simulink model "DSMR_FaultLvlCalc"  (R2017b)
settings: Solver=FixedStepDiscrete  StartTime=0.0  StopTime=10.0  FixedStep=0.02  RelTol=1e-3  EnableMultiTasking=on
undefined symbols (not defined in the file): bin2dec, BMS_DSMR_FaultLvlCalc, Delay, Delay1, DFES_Cls_DFC_638LinCommErr_C, DFES_Cls_DFC_AcDischgFobd_C, DFES_Cls_DFC_AChgFobd_C, DFES_Cls_DFC_AChgHVOffTmt_C, DFES_Cls_DFC_AChgHVOnTmt_C, DFES_Cls_DFC_AChgingErr_C, DFES_Cls_DFC_AChgLckTmt_C, DFES_Cls_DFC_AChgPileRdyTmt_C, DFES_Cls_DFC_AChgRdyPndiTmt_C, DFES_Cls_DFC_AChgRdyTmt_C, DFES_Cls_DFC_AChgS2ClsdTmt_C, DFES_Cls_DFC_AChgUnlckTmt_C, DFES_Cls_DFC_AChrgCnntErr_C, DFES_Cls_DFC_AChrgCurrMish_C, DFES_Cls_DFC_AChrgPortOvrTemp_C, DFES_Cls_DFC_AChrgVoltMish_C, DFES_Cls_DFC_AFEAdcRelatedErr_C, DFES_Cls_DFC_AFECellTempUpdErr_C, DFES_Cls_DFC_AFECellVoltLineOpen_C, DFES_Cls_DFC_AFECellVoltUpdErr_C, DFES_Cls_DFC_AFEComLost_C, DFES_Cls_DFC_AFEDiagModeExitErr_C, DFES_Cls_DFC_AFEGpioLineOpen_C, DFES_Cls_DFC_AFEOtherErr_C, DFES_Cls_DFC_AFEResetFlt_C, DFES_Cls_DFC_AFESampleErr_C, DFES_Cls_DFC_AFESplyFlt_C, DFES_Cls_DFC_AFETempHighFlt_C, DFES_Cls_DFC_APlusChk_C, DFES_Cls_DFC_BalCirOpenFlt_C, DFES_Cls_DFC_BalCirShortFlt_C, DFES_Cls_DFC_BalStuckMax_C, DFES_Cls_DFC_BalStuckMin_C, DFES_Cls_DFC_BalTempHighFlt_C, DFES_Cls_DFC_BattCurrMismatchErr_C, DFES_Cls_DFC_BattHVMsgTmt_C, DFES_Cls_DFC_BattSohChk_C, DFES_Cls_DFC_BattTAlrmMax_C, DFES_Cls_DFC_BattTAlrmMin_C, DFES_Cls_DFC_BattTCnstMax_C, DFES_Cls_DFC_BattTempVldMax_C, DFES_Cls_DFC_BattTempVldMin_C, DFES_Cls_DFC_BattTFaultMax_C, DFES_Cls_DFC_BattTFaultMin_C, DFES_Cls_DFC_BattTGradtMax_C, DFES_Cls_DFC_BattTHopMax_C, DFES_Cls_DFC_BattTWarnMax_C, DFES_Cls_DFC_BattTWarnMin_C, DFES_Cls_DFC_BattUNpl_C, DFES_Cls_DFC_BattVoltHiMax_C, DFES_Cls_DFC_BattVoltLoMin_C, DFES_Cls_DFC_BattVoltRngErr_C, DFES_Cls_DFC_BattVoltVld_C, DFES_Cls_DFC_BMSSplyPwrAbnToCAB_C, DFES_Cls_DFC_BMSSplyPwrAbnToLem_C, DFES_Cls_DFC_BoardTempTmt_C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
libraries: simulink x535
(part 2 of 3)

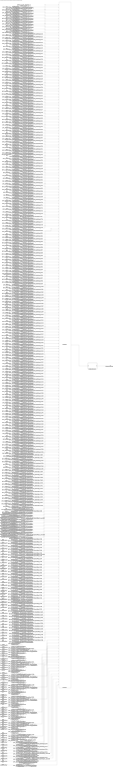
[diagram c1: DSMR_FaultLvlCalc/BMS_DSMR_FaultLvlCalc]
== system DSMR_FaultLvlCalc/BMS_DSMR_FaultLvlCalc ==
  DFC_CurrRngErr : Inport
  DFC_BattVoltRngErr : Inport  Port=2
  DFC_BattHVMsgTmt : Inport  Port=3
  DFC_BusHVMsgTmt : Inport  Port=4
  DFC_638LinCommErr : Inport  Port=5
  DFC_CellTempTmt : Inport  Port=6
  DFC_CellVoltTmt : Inport  Port=7
  DFC_InCanBusOff : Inport  Port=8
  DFC_VeCanBusOff : Inport  Port=9
  DFC_Msg2A3Tmt : Inport  Port=10
  DFC_RcMsg2A3Mis : Inport  Port=11
  DFC_ChkSumMsg2A3Err : Inport  Port=12
  DFC_RcMsg2A5Mis : Inport  Port=13
  DFC_RcMsg2A7Mis : Inport  Port=14
  DFC_CrashNpl : Inport  Port=15
  DFC_FuseNpl : Inport  Port=16
  DFC_Kl30cVoltLoErr : Inport  Port=17
  DFC_PosStuckMax : Inport  Port=18
  DFC_MPosStuckMin : Inport  Port=19
  DFC_MNegStuckMax : Inport  Port=20
  DFC_MNegStuckMin : Inport  Port=21
  DFC_PrStuckMin : Inport  Port=22
  DFC_DChrgPosStuckMax : Inport  Port=23
  DFC_DChrgPosStuckMin : Inport  Port=24
  DFC_DChrgNegStuckMax : Inport  Port=25
  DFC_DChrgNegStuckMin : Inport  Port=26
  DFC_HvPwrUpFail : Inport  Port=27
  DFC_DChrgPwrUpFail : Inport  Port=28
  DFC_BattTAlrmMax : Inport  Port=29
  DFC_BattTFaultMax : Inport  Port=30
  DFC_BattTAlrmMin : Inport  Port=31
  DFC_BattTFaultMin : Inport  Port=32
  DFC_BattTempVldMin : Inport  Port=33
  DFC_BattTCnstMax : Inport  Port=34
  DFC_BattTGradtMax : Inport  Port=35
  DFC_CellVoltAlrmMax : Inport  Port=36
  DFC_CellVoltFaultMax : Inport  Port=37
  DFC_CellVoltFusfMax : Inport  Port=38
  DFC_CellVoltAlrmMin : Inport  Port=39
  DFC_CellVoltFusfMin : Inport  Port=40
  DFC_CellVoltFaultMin : Inport  Port=41
  DFC_CellVoltVldMin : Inport  Port=42
  DFC_CellVoltNpl : Inport  Port=43
  DFC_Msg2E6Tmt : Inport  Port=44
  DFC_RcMsg2E6Mis : Inport  Port=45
  DFC_ChkSumMsg2E6Err : Inport  Port=46
  DFC_RcMsg2E1Mis : Inport  Port=47
  DFC_ChkSumMsg2E1Err : Inport  Port=48
  DFC_DcCanBusOff : Inport  Port=49
  DFC_DChrgTCnntMax : Inport  Port=50
  DFC_ChrgOCNpl : Inport  Port=51
  DFC_DisChOCNpl : Inport  Port=52
  DFC_BattVoltHiMax : Inport  Port=53
  DFC_BattVoltLoMin : Inport  Port=54
  DFC_ThmRnwy : Inport  Port=55
  DFC_AChrgPortOvrTemp : Inport  Port=56
  DFC_CurrOffsPlaus : Inport  Port=57
  DFC_CurrStukPlaus : Inport  Port=58
  DFC_CurrChrgPlaus : Inport  Port=59
  DFC_BattUNpl : Inport  Port=60
  DFC_BattVoltVld : Inport  Port=61
  DFC_PackUNpl : Inport  Port=62
  DFC_PackVoltVld : Inport  Port=63
  DFC_DChrgUNpl : Inport  Port=64
  DFC_DChrgVoltVld : Inport  Port=65
  DFC_BoardTempTmt : Inport  Port=66
  DFC_HvilMax : Inport  Port=67
  DFC_HvilMin : Inport  Port=68
  DFC_HvilSig : Inport  Port=69
  DFC_ChkSumMsg050Err : Inport  Port=70
  DFC_RcMsg050Mis : Inport  Port=71
  DFC_CrashHwNpl : Inport  Port=72
  DFC_IsoChkLv1 : Inport  Port=73
  DFC_IsoChkLv2 : Inport  Port=74
  DFC_InsResValdFault : Inport  Port=75
  DFC_Kl30OutRngErr : Inport  Port=76
  DFC_Kl30VoltLoErr : Inport  Port=77
  DFC_Kl30VoltHiErr : Inport  Port=78
  DFC_EepReadErr : Inport  Port=79
  DFC_BalStuckMax : Inport  Port=80
  DFC_BalStuckMin : Inport  Port=81
  DFC_CSCPwrSpyHiErr : Inport  Port=82
  DFC_CSCPwrSpyLoErr : Inport  Port=83
  DFC_CmcBordOTMax : Inport  Port=84
  DFC_BattTWarnMax : Inport  Port=85
  DFC_BattTWarnMin : Inport  Port=86
  DFC_BattTempVldMax : Inport  Port=87
  DFC_BattTHopMax : Inport  Port=88
  DFC_CellVoltRngHiErr : Inport  Port=89
  DFC_CellVoltRngLoErr : Inport  Port=90
  DFC_CellVoltWarnMax : Inport  Port=91
  DFC_CellVoltWarnMin : Inport  Port=92
  DFC_CellVoltVldMax : Inport  Port=93
  DFC_AChrgCurrMish : Inport  Port=94
  DFC_DChrgCurrMish : Inport  Port=95
  DFC_DChrgLowTempCurrMish : Inport  Port=96
  DFC_AChrgVoltMish : Inport  Port=97
  DFC_DChrgVoltMish : Inport  Port=98
  DFC_DChrgBattTMin : Inport  Port=99
  DFC_CC2Chk : Inport  Port=100
  DFC_APlusChk : Inport  Port=101
  DFC_DChrgMsgTmt : Inport  Port=102
  DFC_DChrgTNegElecMax : Inport  Port=103
  DFC_DChrgTNegElecMin : Inport  Port=104
  DFC_DChrgTNegElecSig : Inport  Port=105
  DFC_DChrgTPosElecMax : Inport  Port=106
  DFC_DChrgTPosElecMin : Inport  Port=107
  DFC_DChrgTPosElecSig : Inport  Port=108
  DFC_CcuSelfChkErr : Inport  Port=109
  DFC_ChrgOCMin : Inport  Port=110
  DFC_ChrgOCMax : Inport  Port=111
  DFC_DisChOCMin : Inport  Port=112
  DFC_DisChOCMax : Inport  Port=113
  DFC_SocRngLoMax : Inport  Port=114
  DFC_SocRngLoMin : Inport  Port=115
  DFC_SocRngHiMax : Inport  Port=116
  DFC_SocRngHiMin : Inport  Port=117
  DFC_InClntOverTmp : Inport  Port=118
  DFC_OutClntOverTmp : Inport  Port=119
  DFC_ClntDsTElecMax : Inport  Port=120
  DFC_ClntDsTElecMin : Inport  Port=121
  DFC_ClntDsTElecSig : Inport  Port=122
  DFC_ClntUsTElecMax : Inport  Port=123
  DFC_ClntUsTElecMin : Inport  Port=124
  DFC_ClntUsTElecSig : Inport  Port=125
  DFC_CoolPerfPlaus : Inport  Port=126
  DFC_HtgPerfPlaus : Inport  Port=127
  DFC_DChrgFobd : Inport  Port=128
  DFC_DChrgHvOnFail : Inport  Port=129
  DFC_AChgHVOnTmt : Inport  Port=130
  DFC_AChgHVOffTmt : Inport  Port=131
  DFC_AChgS2ClsdTmt : Inport  Port=132
  DFC_DChrgStakeErr : Inport  Port=133
  DFC_DChrgStkVoltErr : Inport  Port=134
  DFC_DChrgStkCurrErr : Inport  Port=135
  DFC_AChgPileRdyTmt : Inport  Port=136
  DFC_DChrgCHMTmt : Inport  Port=137
  DFC_DChrgCRMTmt : Inport  Port=138
  DFC_DChrgCMLTmt : Inport  Port=139
  DFC_DChrgCROTmt : Inport  Port=140
  DFC_DChrgCCSTmt : Inport  Port=141
  DFC_DChrgCSTTmt : Inport  Port=142
  DFC_DChrgCSDTmt : Inport  Port=143
  DFC_DChrgParaChk : Inport  Port=144
  DFC_DChrgCableChk : Inport  Port=145
  DFC_DChrgSLACTOut : Inport  Port=146
  DFC_DChrgCnntErr : Inport  Port=147
  DFC_DChrgLckErr : Inport  Port=148
  DFC_AChrgCnntErr : Inport  Port=149
  DFC_AChgLckTmt : Inport  Port=150
  DFC_AChgRdyPndiTmt : Inport  Port=151
  DFC_AChgRdyTmt : Inport  Port=152
  DFC_AChgingErr : Inport  Port=153
  DFC_AChgUnlckTmt : Inport  Port=154
  DFC_AChgFobd : Inport  Port=155
  DFC_SocValJmp : Inport  Port=156
  DFC_ChrgCmuLost : Inport  Port=157
  DFC_DisChrgCmuLost : Inport  Port=158
  DFC_Msg130Tmt : Inport  Port=159
  DFC_Msg2E1Tmt : Inport  Port=160
  DFC_Msg2EBTmt : Inport  Port=161
  DFC_MsgCABTmt : Inport  Port=162
  DFC_Msg0B5Tmt : Inport  Port=163
  DFC_ObcTmt : Inport  Port=164
  DFC_VcuTmt : Inport  Port=165
  DFC_Msg2A7Tmt : Inport  Port=166
  DFC_Msg2A5Tmt : Inport  Port=167
  DFC_Msg2ADTmt : Inport  Port=168
  DFC_Msg2BBTmt : Inport  Port=169
  DFC_Msg2DFTmt : Inport  Port=170
  DFC_Msg3AATmt : Inport  Port=171
  DFC_Msg050Tmt : Inport  Port=172
  DFC_Msg2F1Tmt : Inport  Port=173
  DFC_Msg195Tmt : Inport  Port=174
  DFC_Msg37FTmt : Inport  Port=175
  DFC_Msg28CTmt : Inport  Port=176
  DFC_Msg17DTmt : Inport  Port=177
  DFC_HwCurrElecSCG : Inport  Port=178
  DFC_HwCurrElecSCP : Inport  Port=179
  DFC_CABErr : Inport  Port=180
  DFC_BattCurrMismatchErr : Inport  Port=181
  GaCFM_AFEComLost_flg : Inport  Port=182
  GaCFM_AFECellVoltUpdErr_flg : Inport  Port=183
  GaCFM_AFECellTempUpdErr_flg : Inport  Port=184
  GaCFM_AFESampleErr_flg : Inport  Port=185
  GaCFM_AFECellVoltLineOpen_flg : Inport  Port=186
  GaCFM_AFEGpioLineOpen_flg : Inport  Port=187
  GaCFM_AFEAdcRelatedErr_flg : Inport  Port=188
  GaCFM_AFEDiagModeExitErr_flg : Inport  Port=189
  GaCFM_AFEOtherErr_flg : Inport  Port=190
  DFC_AcDischgFobd : Inport  Port=191
  DFC_BalCirOpenFlt : Inport  Port=192
  DFC_BalCirShortFlt : Inport  Port=193
  DFC_BalTempHighFlt : Inport  Port=194
  DFC_HVSmplComFlt : Inport  Port=195
  DFC_HVSmplSigErr : Inport  Port=196
  DFC_HVSmplSplyFlt : Inport  Port=197
  DFC_CABVoltOutOfRng : Inport  Port=198
  DFC_CABDevFlt : Inport  Port=199
  DFC_BMSSplyPwrAbnToLem : Inport  Port=200
  DFC_BMSSplyPwrAbnToCAB : Inport  Port=201
  DFC_NVMReadError : Inport  Port=202
  DFC_KL30Shutdown : Inport  Port=203
  DFC_MCUResetFlt : Inport  Port=204
  DFC_BattSohChk : Inport  Port=205
  DFC_CalCANBusOff : Inport  Port=206
  DFC_ThmRnwyWarn : Inport  Port=207
  DFC_PchgOvrCurrFlt : Inport  Port=208
  DFC_SBCSplyPwrOvrVolt : Inport  Port=209
  DFC_SBCSplyPwrUnderVolt : Inport  Port=210
  DFC_SBCSplyPwrOvrCurr : Inport  Port=211
  DFC_CrashChkHwFrqAbnorm : Inport  Port=212
  DFC_CrashChkHwDutyAbnorm : Inport  Port=213
  DFC_AFETempHighFlt : Inport  Port=214
  DFC_EVCCDevFlt : Inport  Port=215
  DFC_EVCCSplyPwrFlt : Inport  Port=216
  DFC_EVCCVehComFlt : Inport  Port=217
  DFC_EVCCPileComFlt : Inport  Port=218
  DFC_EVCCVehHwFlt : Inport  Port=219
  DFC_EVCCPileHwFlt : Inport  Port=220
  DFC_IsoS1SwStuckOpen : Inport  Port=221
  DFC_IsoS1SwStuckClsd : Inport  Port=222
  DFC_IsoS2SwStuckOpen : Inport  Port=223
  DFC_IsoS2SwStuckClsd : Inport  Port=224
  DFC_IsoS3SwStuckOpen : Inport  Port=225
  DFC_IsoS3SwStuckClsd : Inport  Port=226
  DFC_AFEResetFlt : Inport  Port=227
  DFC_AFESplyFlt : Inport  Port=228
  DFC_PreHeatErr : Inport  Port=229
  DFC_PreHeatVcuReqTmt : Inport  Port=230
  DFC_PreHeatObcStatusErr : Inport  Port=231
  DFC_PreHeatPtcErr : Inport  Port=232
  DFC_MPosRlyDrvScb : Inport  Port=233
  DFC_MPosRlyDrvScg : Inport  Port=234
  DFC_MPosRlyDrvOL : Inport  Port=235
  DFC_MposRlyDrvOvrCurr : Inport  Port=236
  DFC_MPosRlyDrvFault : Inport  Port=237
  DFC_MNegRlyDrvScb : Inport  Port=238
  DFC_MNegRlyDrvScg : Inport  Port=239
  DFC_MNegRlyDrvOL : Inport  Port=240
  DFC_MNegRlyDrvOvrCurr : Inport  Port=241
  DFC_MNegRlyDrvFault : Inport  Port=242
  DFC_DcPosRlyDrvScb : Inport  Port=243
  DFC_DcPosRlyDrvScg : Inport  Port=244
  DFC_DcPosRlyDrvOL : Inport  Port=245
  DFC_DChrgPosRlyDrvOvrCurr : Inport  Port=246
  DFC_DcPosRlyDrvFault : Inport  Port=247
  DFC_DcNegRlyDrvScb : Inport  Port=248
  DFC_DcNegRlyDrvScg : Inport  Port=249
  DFC_DcNegRlyDrvOL : Inport  Port=250
  DFC_DChrgNegRlyDrvOvrCurr : Inport  Port=251
  DFC_DcNegRlyDrvFault : Inport  Port=252
  DFC_PreRlyDrvScb : Inport  Port=253
  DFC_PreRlyDrvScg : Inport  Port=254
  DFC_PreRlyDrvOL : Inport  Port=255
  DFC_PrRlyDrvOvrCurr : Inport  Port=256
  DFC_CellTAlrmMax : Inport  Port=257
  DFC_CellTFaultMax : Inport  Port=258
  DFC_CellTAlrmMin : Inport  Port=259
  DFC_CellTFaultMin : Inport  Port=260
  DFC_CellTempVldMin : Inport  Port=261
  DFC_CellTCnstMax : Inport  Port=262
  DFC_CellTGradtMax : Inport  Port=263
  DFC_CellTWarnMax : Inport  Port=264
  DFC_CellTWarnMin : Inport  Port=265
  DFC_CellTempVldMax : Inport  Port=266
  DFC_CellTHopMax : Inport  Port=267
  DFC_TwoCurrSnsrFlt : Inport  Port=268
  DFC_ThmRnwyAlarm : Inport  Port=269
  DFC_ChkSumMsg2A5Err : Inport  Port=270
  DFC_ChkSumMsg2A7Err : Inport  Port=271
  DFC_DchrgIsoChkLv1 : Inport  Port=272
  DFC_DchrgIsoChkLv2 : Inport  Port=273
  DFC_HVOffIsoChkLv1 : Inport  Port=274
  DFC_HVOffIsoChkLv2 : Inport  Port=275
  DFC_PackCrntSaf : Inport  Port=276
  DFC_BattUNpl_{1..267} (267 alike) : simulink/Logic and Bit Operations/Bitwise Operator  logicop=AND  UseBitMask=on  BitMask=bin2dec('00011000')  BitMaskRealWorld=Stored Integer
  DFC_BattUNpl_1_compare{,1..266} (267 alike) : simulink/Logic and Bit Operations/Compare To Constant  relop===  const=24  OutDataTypeStr=boolean
  DFC_BattUNpl_applied{,1..243} (244 alike) : Switch  Criteria=u2 > Threshold
  DFES_Cls_DFC_BattUNpl_C : Constant  Value=DFES_Cls_DFC_CurrRngErr_C
  DFES_Cls_DFC_BattUNpl_C1 : Constant  Value=DFES_Cls_DFC_BattVoltRngErr_C
  DFES_Cls_DFC_BattUNpl_C10 : Constant  Value=DFES_Cls_DFC_RcMsg2A3Mis_C
  DFES_Cls_DFC_BattUNpl_C100 : Constant  Value=DFES_Cls_DFC_APlusChk_C
  DFES_Cls_DFC_BattUNpl_C101 : Constant  Value=DFES_Cls_DFC_DChrgMsgTmt_C
  DFES_Cls_DFC_BattUNpl_C102 : Constant  Value=DFES_Cls_DFC_DChrgTNegElecMax_C
  DFES_Cls_DFC_BattUNpl_C103 : Constant  Value=DFES_Cls_DFC_DChrgTNegElecMin_C
  DFES_Cls_DFC_BattUNpl_C104 : Constant  Value=DFES_Cls_DFC_DChrgTNegElecSig_C
  DFES_Cls_DFC_BattUNpl_C105 : Constant  Value=DFES_Cls_DFC_DChrgTPosElecMax_C
  DFES_Cls_DFC_BattUNpl_C106 : Constant  Value=DFES_Cls_DFC_DChrgTPosElecMin_C
  DFES_Cls_DFC_BattUNpl_C107 : Constant  Value=DFES_Cls_DFC_DChrgTPosElecSig_C
  DFES_Cls_DFC_BattUNpl_C108 : Constant  Value=DFES_Cls_DFC_CcuSelfChkErr_C
  DFES_Cls_DFC_BattUNpl_C109 : Constant  Value=DFES_Cls_DFC_ChrgOCMin_C
  DFES_Cls_DFC_BattUNpl_C11 : Constant  Value=DFES_Cls_DFC_ChkSumMsg2A3Err_C
  DFES_Cls_DFC_BattUNpl_C110 : Constant  Value=DFES_Cls_DFC_ChrgOCMax_C
  DFES_Cls_DFC_BattUNpl_C111 : Constant  Value=DFES_Cls_DFC_DisChOCMin_C
  DFES_Cls_DFC_BattUNpl_C112 : Constant  Value=DFES_Cls_DFC_DisChOCMax_C
  DFES_Cls_DFC_BattUNpl_C113 : Constant  Value=DFES_Cls_DFC_SocRngLoMax_C
  DFES_Cls_DFC_BattUNpl_C114 : Constant  Value=DFES_Cls_DFC_SocRngLoMin_C
  DFES_Cls_DFC_BattUNpl_C115 : Constant  Value=DFES_Cls_DFC_SocRngHiMax_C
  DFES_Cls_DFC_BattUNpl_C116 : Constant  Value=DFES_Cls_DFC_SocRngHiMin_C
  DFES_Cls_DFC_BattUNpl_C117 : Constant  Value=DFES_Cls_DFC_InClntOverTmp_C
  DFES_Cls_DFC_BattUNpl_C118 : Constant  Value=DFES_Cls_DFC_OutClntOverTmp_C
  DFES_Cls_DFC_BattUNpl_C119 : Constant  Value=DFES_Cls_DFC_ClntDsTElecMax_C
  DFES_Cls_DFC_BattUNpl_C12 : Constant  Value=DFES_Cls_DFC_RcMsg2A5Mis_C
  DFES_Cls_DFC_BattUNpl_C120 : Constant  Value=DFES_Cls_DFC_ClntDsTElecMin_C
  DFES_Cls_DFC_BattUNpl_C121 : Constant  Value=DFES_Cls_DFC_ClntDsTElecSig_C
  DFES_Cls_DFC_BattUNpl_C122 : Constant  Value=DFES_Cls_DFC_ClntUsTElecMax_C
  DFES_Cls_DFC_BattUNpl_C123 : Constant  Value=DFES_Cls_DFC_ClntUsTElecMin_C
  DFES_Cls_DFC_BattUNpl_C124 : Constant  Value=DFES_Cls_DFC_ClntUsTElecSig_C
  DFES_Cls_DFC_BattUNpl_C125 : Constant  Value=DFES_Cls_DFC_CoolPerfPlaus_C
  DFES_Cls_DFC_BattUNpl_C126 : Constant  Value=DFES_Cls_DFC_HtgPerfPlaus_C
  DFES_Cls_DFC_BattUNpl_C127 : Constant  Value=DFES_Cls_DFC_DChrgFobd_C
  DFES_Cls_DFC_BattUNpl_C128 : Constant  Value=DFES_Cls_DFC_DChrgHvOnFail_C
  DFES_Cls_DFC_BattUNpl_C129 : Constant  Value=DFES_Cls_DFC_AChgHVOnTmt_C
  DFES_Cls_DFC_BattUNpl_C13 : Constant  Value=DFES_Cls_DFC_RcMsg2A7Mis_C
  DFES_Cls_DFC_BattUNpl_C130 : Constant  Value=DFES_Cls_DFC_AChgHVOffTmt_C
  DFES_Cls_DFC_BattUNpl_C131 : Constant  Value=DFES_Cls_DFC_AChgS2ClsdTmt_C
  DFES_Cls_DFC_BattUNpl_C132 : Constant  Value=DFES_Cls_DFC_DChrgStakeErr_C
  DFES_Cls_DFC_BattUNpl_C133 : Constant  Value=DFES_Cls_DFC_DChrgStkVoltErr_C
  DFES_Cls_DFC_BattUNpl_C134 : Constant  Value=DFES_Cls_DFC_DChrgStkCurrErr_C
  DFES_Cls_DFC_BattUNpl_C135 : Constant  Value=DFES_Cls_DFC_AChgPileRdyTmt_C
  DFES_Cls_DFC_BattUNpl_C136 : Constant  Value=DFES_Cls_DFC_DChrgCHMTmt_C
  DFES_Cls_DFC_BattUNpl_C137 : Constant  Value=DFES_Cls_DFC_DChrgCRMTmt_C
  DFES_Cls_DFC_BattUNpl_C138 : Constant  Value=DFES_Cls_DFC_DChrgCMLTmt_C
  DFES_Cls_DFC_BattUNpl_C139 : Constant  Value=DFES_Cls_DFC_DChrgCROTmt_C
  DFES_Cls_DFC_BattUNpl_C14 : Constant  Value=DFES_Cls_DFC_CrashNpl_C
  DFES_Cls_DFC_BattUNpl_C140 : Constant  Value=DFES_Cls_DFC_DChrgCCSTmt_C
  DFES_Cls_DFC_BattUNpl_C141 : Constant  Value=DFES_Cls_DFC_DChrgCSTTmt_C
  DFES_Cls_DFC_BattUNpl_C142 : Constant  Value=DFES_Cls_DFC_DChrgCSDTmt_C
  DFES_Cls_DFC_BattUNpl_C143 : Constant  Value=DFES_Cls_DFC_DChrgParaChk_C
  DFES_Cls_DFC_BattUNpl_C144 : Constant  Value=DFES_Cls_DFC_DChrgCableChk_C
  DFES_Cls_DFC_BattUNpl_C145 : Constant  Value=DFES_Cls_DFC_DChrgSLACTOut_C
  DFES_Cls_DFC_BattUNpl_C146 : Constant  Value=DFES_Cls_DFC_DChrgCnntErr_C
  DFES_Cls_DFC_BattUNpl_C147 : Constant  Value=DFES_Cls_DFC_DChrgLckErr_C
  DFES_Cls_DFC_BattUNpl_C148 : Constant  Value=DFES_Cls_DFC_AChrgCnntErr_C
  DFES_Cls_DFC_BattUNpl_C149 : Constant  Value=DFES_Cls_DFC_AChgLckTmt_C
  DFES_Cls_DFC_BattUNpl_C15 : Constant  Value=DFES_Cls_DFC_FuseNpl_C
  DFES_Cls_DFC_BattUNpl_C150 : Constant  Value=DFES_Cls_DFC_AChgRdyPndiTmt_C
  DFES_Cls_DFC_BattUNpl_C151 : Constant  Value=DFES_Cls_DFC_AChgRdyTmt_C
  DFES_Cls_DFC_BattUNpl_C152 : Constant  Value=DFES_Cls_DFC_AChgingErr_C
  DFES_Cls_DFC_BattUNpl_C153 : Constant  Value=DFES_Cls_DFC_AChgUnlckTmt_C
  DFES_Cls_DFC_BattUNpl_C154 : Constant  Value=DFES_Cls_DFC_AChgFobd_C
  DFES_Cls_DFC_BattUNpl_C155 : Constant  Value=DFES_Cls_DFC_SocValJmp_C
  DFES_Cls_DFC_BattUNpl_C156 : Constant  Value=DFES_Cls_DFC_ChrgCmuLost_C
  DFES_Cls_DFC_BattUNpl_C157 : Constant  Value=DFES_Cls_DFC_DisChrgCmuLost_C
  DFES_Cls_DFC_BattUNpl_C158 : Constant  Value=DFES_Cls_DFC_Msg130Tmt_C
  DFES_Cls_DFC_BattUNpl_C159 : Constant  Value=DFES_Cls_DFC_Msg2E1Tmt_C
  DFES_Cls_DFC_BattUNpl_C16 : Constant  Value=DFES_Cls_DFC_Kl30cVoltLoErr_C
  DFES_Cls_DFC_BattUNpl_C160 : Constant  Value=DFES_Cls_DFC_Msg2EBTmt_C
  DFES_Cls_DFC_BattUNpl_C161 : Constant  Value=DFES_Cls_DFC_MsgCABTmt_C
  DFES_Cls_DFC_BattUNpl_C162 : Constant  Value=DFES_Cls_DFC_Msg0B5Tmt_C
  DFES_Cls_DFC_BattUNpl_C163 : Constant  Value=DFES_Cls_DFC_ObcTmt_C
  DFES_Cls_DFC_BattUNpl_C164 : Constant  Value=DFES_Cls_DFC_VcuTmt_C
  DFES_Cls_DFC_BattUNpl_C165 : Constant  Value=DFES_Cls_DFC_Msg2A7Tmt_C
  DFES_Cls_DFC_BattUNpl_C166 : Constant  Value=DFES_Cls_DFC_Msg2A5Tmt_C
  DFES_Cls_DFC_BattUNpl_C167 : Constant  Value=DFES_Cls_DFC_Msg2ADTmt_C
  DFES_Cls_DFC_BattUNpl_C168 : Constant  Value=DFES_Cls_DFC_Msg2BBTmt_C
  DFES_Cls_DFC_BattUNpl_C169 : Constant  Value=DFES_Cls_DFC_Msg2DFTmt_C
  DFES_Cls_DFC_BattUNpl_C17 : Constant  Value=DFES_Cls_DFC_PosStuckMax_C
  DFES_Cls_DFC_BattUNpl_C170 : Constant  Value=DFES_Cls_DFC_Msg3AATmt_C
  DFES_Cls_DFC_BattUNpl_C171 : Constant  Value=DFES_Cls_DFC_Msg050Tmt_C
  DFES_Cls_DFC_BattUNpl_C172 : Constant  Value=DFES_Cls_DFC_Msg2F1Tmt_C
  DFES_Cls_DFC_BattUNpl_C173 : Constant  Value=DFES_Cls_DFC_Msg37FTmt_C
  DFES_Cls_DFC_BattUNpl_C174 : Constant  Value=DFES_Cls_DFC_Msg28CTmt_C
  DFES_Cls_DFC_BattUNpl_C175 : Constant  Value=DFES_Cls_DFC_Msg17DTmt_C
  DFES_Cls_DFC_BattUNpl_C176 : Constant  Value=DFES_Cls_DFC_HwCurrElecSCG_C
  DFES_Cls_DFC_BattUNpl_C177 : Constant  Value=DFES_Cls_DFC_HwCurrElecSCP_C
  DFES_Cls_DFC_BattUNpl_C178 : Constant  Value=DFES_Cls_DFC_CABErr_C
  DFES_Cls_DFC_BattUNpl_C179 : Constant  Value=DFES_Cls_DFC_BattCurrMismatchErr_C
  DFES_Cls_DFC_BattUNpl_C18 : Constant  Value=DFES_Cls_DFC_MPosStuckMin_C
  DFES_Cls_DFC_BattUNpl_C180 : Constant  Value=DFES_Cls_DFC_Msg195Tmt_C
  DFES_Cls_DFC_BattUNpl_C181 : Constant  Value=DFES_Cls_DFC_AFEComLost_C
  DFES_Cls_DFC_BattUNpl_C182 : Constant  Value=DFES_Cls_DFC_AFECellVoltUpdErr_C
  DFES_Cls_DFC_BattUNpl_C183 : Constant  Value=DFES_Cls_DFC_AFECellTempUpdErr_C
  DFES_Cls_DFC_BattUNpl_C184 : Constant  Value=DFES_Cls_DFC_AFESampleErr_C
  DFES_Cls_DFC_BattUNpl_C185 : Constant  Value=DFES_Cls_DFC_AFECellVoltLineOpen_C
  DFES_Cls_DFC_BattUNpl_C186 : Constant  Value=DFES_Cls_DFC_AFEGpioLineOpen_C
  DFES_Cls_DFC_BattUNpl_C187 : Constant  Value=DFES_Cls_DFC_AFEAdcRelatedErr_C
  DFES_Cls_DFC_BattUNpl_C188 : Constant  Value=DFES_Cls_DFC_AFEDiagModeExitErr_C
  DFES_Cls_DFC_BattUNpl_C189 : Constant  Value=DFES_Cls_DFC_AFEOtherErr_C
  DFES_Cls_DFC_BattUNpl_C19 : Constant  Value=DFES_Cls_DFC_MNegStuckMax_C
  DFES_Cls_DFC_BattUNpl_C190 : Constant  Value=DFES_Cls_DFC_AcDischgFobd_C
  DFES_Cls_DFC_BattUNpl_C191 : Constant  Value=DFES_Cls_DFC_BalCirOpenFlt_C
  DFES_Cls_DFC_BattUNpl_C192 : Constant  Value=DFES_Cls_DFC_BalCirShortFlt_C
  DFES_Cls_DFC_BattUNpl_C193 : Constant  Value=DFES_Cls_DFC_BalTempHighFlt_C
  DFES_Cls_DFC_BattUNpl_C194 : Constant  Value=DFES_Cls_DFC_HVSmplComFlt_C
  DFES_Cls_DFC_BattUNpl_C195 : Constant  Value=DFES_Cls_DFC_HVSmplSigErr_C
  DFES_Cls_DFC_BattUNpl_C196 : Constant  Value=DFES_Cls_DFC_HVSmplSplyFlt_C
  DFES_Cls_DFC_BattUNpl_C197 : Constant  Value=DFES_Cls_DFC_CABVoltOutOfRng_C
  DFES_Cls_DFC_BattUNpl_C198 : Constant  Value=DFES_Cls_DFC_CABDevFlt_C
  DFES_Cls_DFC_BattUNpl_C199 : Constant  Value=DFES_Cls_DFC_BMSSplyPwrAbnToLem_C
  DFES_Cls_DFC_BattUNpl_C2 : Constant  Value=DFES_Cls_DFC_BattHVMsgTmt_C
  DFES_Cls_DFC_BattUNpl_C20 : Constant  Value=DFES_Cls_DFC_MNegStuckMin_C
  DFES_Cls_DFC_BattUNpl_C200 : Constant  Value=DFES_Cls_DFC_BMSSplyPwrAbnToCAB_C
  DFES_Cls_DFC_BattUNpl_C201 : Constant  Value=DFES_Cls_DFC_NVMReadError_C
  DFES_Cls_DFC_BattUNpl_C202 : Constant  Value=DFES_Cls_DFC_KL30Shutdown_C
  DFES_Cls_DFC_BattUNpl_C203 : Constant  Value=DFES_Cls_DFC_MCUResetFlt_C
  DFES_Cls_DFC_BattUNpl_C204 : Constant  Value=DFES_Cls_DFC_BattSohChk_C
  DFES_Cls_DFC_BattUNpl_C205 : Constant  Value=DFES_Cls_DFC_CalCANBusOff_C
  DFES_Cls_DFC_BattUNpl_C206 : Constant  Value=DFES_Cls_DFC_ThmRnwyWarn_C
  DFES_Cls_DFC_BattUNpl_C207 : Constant  Value=DFES_Cls_DFC_PchgOvrCurrFlt_C
  DFES_Cls_DFC_BattUNpl_C208 : Constant  Value=DFES_Cls_DFC_SBCSplyPwrOvrVolt_C
  DFES_Cls_DFC_BattUNpl_C209 : Constant  Value=DFES_Cls_DFC_SBCSplyPwrUnderVolt_C
  DFES_Cls_DFC_BattUNpl_C21 : Constant  Value=DFES_Cls_DFC_PrStuckMin_C
  DFES_Cls_DFC_BattUNpl_C210 : Constant  Value=DFES_Cls_DFC_SBCSplyPwrOvrCurr_C
  DFES_Cls_DFC_BattUNpl_C211 : Constant  Value=DFES_Cls_DFC_CrashChkHwFrqAbnorm_C
  DFES_Cls_DFC_BattUNpl_C212 : Constant  Value=DFES_Cls_DFC_AFETempHighFlt_C
  DFES_Cls_DFC_BattUNpl_C213 : Constant  Value=DFES_Cls_DFC_CrashChkHwDutyAbnorm_C
  DFES_Cls_DFC_BattUNpl_C214 : Constant  Value=DFES_Cls_DFC_EVCCFlt_C
  DFES_Cls_DFC_BattUNpl_C215 : Constant  Value=DFES_Cls_DFC_IsoSwFlt_C
  DFES_Cls_DFC_BattUNpl_C216 : Constant  Value=DFES_Cls_DFC_AFEResetFlt_C
  DFES_Cls_DFC_BattUNpl_C217 : Constant  Value=DFES_Cls_DFC_AFESplyFlt_C
  DFES_Cls_DFC_BattUNpl_C218 : Constant  Value=DFES_Cls_DFC_PreHeatFlt_C
  DFES_Cls_DFC_BattUNpl_C219 : Constant  Value=DFES_Cls_DFC_MPosRlyDrv_C
  DFES_Cls_DFC_BattUNpl_C22 : Constant  Value=DFES_Cls_DFC_DChrgPosStuckMax_C
  DFES_Cls_DFC_BattUNpl_C220 : Constant  Value=DFES_Cls_DFC_MNegRlyDrv_C
  DFES_Cls_DFC_BattUNpl_C221 : Constant  Value=DFES_Cls_DFC_DCPosRlyDrv_C
  DFES_Cls_DFC_BattUNpl_C222 : Constant  Value=DFES_Cls_DFC_DCNegRlyDrv_C
  DFES_Cls_DFC_BattUNpl_C223 : Constant  Value=DFES_Cls_DFC_PrRlyDrv_C
  DFES_Cls_DFC_BattUNpl_C224 : Constant  Value=DFES_Cls_DFC_CellTAlrmMax_C
  DFES_Cls_DFC_BattUNpl_C225 : Constant  Value=DFES_Cls_DFC_CellTFaultMax_C
  DFES_Cls_DFC_BattUNpl_C226 : Constant  Value=DFES_Cls_DFC_CellTAlrmMin_C
  DFES_Cls_DFC_BattUNpl_C227 : Constant  Value=DFES_Cls_DFC_CellTFaultMin_C
  DFES_Cls_DFC_BattUNpl_C228 : Constant  Value=DFES_Cls_DFC_CellTempVldMin_C
  DFES_Cls_DFC_BattUNpl_C229 : Constant  Value=DFES_Cls_DFC_CellTCnstMax_C
  DFES_Cls_DFC_BattUNpl_C23 : Constant  Value=DFES_Cls_DFC_DChrgPosStuckMin_C
  DFES_Cls_DFC_BattUNpl_C230 : Constant  Value=DFES_Cls_DFC_CellTGradtMax_C
  DFES_Cls_DFC_BattUNpl_C231 : Constant  Value=DFES_Cls_DFC_CellTWarnMax_C
  DFES_Cls_DFC_BattUNpl_C232 : Constant  Value=DFES_Cls_DFC_CellTWarnMin_C
  DFES_Cls_DFC_BattUNpl_C233 : Constant  Value=DFES_Cls_DFC_CellTempVldMax_C
  DFES_Cls_DFC_BattUNpl_C234 : Constant  Value=DFES_Cls_DFC_CellTHopMax_C
  DFES_Cls_DFC_BattUNpl_C235 : Constant  Value=DFES_Cls_DFC_TwoCurrSnsrFlt_C
  DFES_Cls_DFC_BattUNpl_C236 : Constant  Value=DFES_Cls_DFC_ThmRnwyAlarm_C
  DFES_Cls_DFC_BattUNpl_C237 : Constant  Value=DFES_Cls_DFC_ChkSumMsg2A5Err_C
  DFES_Cls_DFC_BattUNpl_C238 : Constant  Value=DFES_Cls_DFC_ChkSumMsg2A7Err_C
  DFES_Cls_DFC_BattUNpl_C239 : Constant  Value=DFES_Cls_DFC_DchrgIsoChkLv1_C
  DFES_Cls_DFC_BattUNpl_C24 : Constant  Value=DFES_Cls_DFC_DChrgNegStuckMax_C
  DFES_Cls_DFC_BattUNpl_C240 : Constant  Value=DFES_Cls_DFC_DchrgIsoChkLv2_C
  DFES_Cls_DFC_BattUNpl_C241 : Constant  Value=DFES_Cls_DFC_HVOffIsoChkLv1_C
  DFES_Cls_DFC_BattUNpl_C242 : Constant  Value=DFES_Cls_DFC_HVOffIsoChkLv2_C
  DFES_Cls_DFC_BattUNpl_C243 : Constant  Value=DFES_Cls_DFC_PackCrntSaf_C
  DFES_Cls_DFC_BattUNpl_C25 : Constant  Value=DFES_Cls_DFC_DChrgNegStuckMin_C
  DFES_Cls_DFC_BattUNpl_C26 : Constant  Value=DFES_Cls_DFC_HvPwrUpFail_C
  DFES_Cls_DFC_BattUNpl_C27 : Constant  Value=DFES_Cls_DFC_DChrgPwrUpFail_C
  DFES_Cls_DFC_BattUNpl_C28 : Constant  Value=DFES_Cls_DFC_BattTAlrmMax_C
  DFES_Cls_DFC_BattUNpl_C29 : Constant  Value=DFES_Cls_DFC_BattTFaultMax_C
  DFES_Cls_DFC_BattUNpl_C3 : Constant  Value=DFES_Cls_DFC_BusHVMsgTmt_C
  DFES_Cls_DFC_BattUNpl_C30 : Constant  Value=DFES_Cls_DFC_BattTAlrmMin_C
  DFES_Cls_DFC_BattUNpl_C31 : Constant  Value=DFES_Cls_DFC_BattTFaultMin_C
  DFES_Cls_DFC_BattUNpl_C32 : Constant  Value=DFES_Cls_DFC_BattTempVldMin_C
  DFES_Cls_DFC_BattUNpl_C33 : Constant  Value=DFES_Cls_DFC_BattTCnstMax_C
  DFES_Cls_DFC_BattUNpl_C34 : Constant  Value=DFES_Cls_DFC_BattTGradtMax_C
  DFES_Cls_DFC_BattUNpl_C35 : Constant  Value=DFES_Cls_DFC_CellVoltAlrmMax_C
  DFES_Cls_DFC_BattUNpl_C36 : Constant  Value=DFES_Cls_DFC_CellVoltFaultMax_C
  DFES_Cls_DFC_BattUNpl_C37 : Constant  Value=DFES_Cls_DFC_CellVoltFusfMax_C
  DFES_Cls_DFC_BattUNpl_C38 : Constant  Value=DFES_Cls_DFC_CellVoltAlrmMin_C
  DFES_Cls_DFC_BattUNpl_C39 : Constant  Value=DFES_Cls_DFC_CellVoltFusfMin_C
  DFES_Cls_DFC_BattUNpl_C4 : Constant  Value=DFES_Cls_DFC_638LinCommErr_C
  DFES_Cls_DFC_BattUNpl_C40 : Constant  Value=DFES_Cls_DFC_CellVoltFaultMin_C
  DFES_Cls_DFC_BattUNpl_C41 : Constant  Value=DFES_Cls_DFC_CellVoltVldMin_C
  DFES_Cls_DFC_BattUNpl_C42 : Constant  Value=DFES_Cls_DFC_CellVoltNpl_C
  DFES_Cls_DFC_BattUNpl_C43 : Constant  Value=DFES_Cls_DFC_Msg2E6Tmt_C
  DFES_Cls_DFC_BattUNpl_C44 : Constant  Value=DFES_Cls_DFC_RcMsg2E6Mis_C
  DFES_Cls_DFC_BattUNpl_C45 : Constant  Value=DFES_Cls_DFC_ChkSumMsg2E6Err_C
  DFES_Cls_DFC_BattUNpl_C46 : Constant  Value=DFES_Cls_DFC_RcMsg2E1Mis_C
  DFES_Cls_DFC_BattUNpl_C47 : Constant  Value=DFES_Cls_DFC_ChkSumMsg2E1Err_C
  DFES_Cls_DFC_BattUNpl_C48 : Constant  Value=DFES_Cls_DFC_DcCanBusOff_C
  DFES_Cls_DFC_BattUNpl_C49 : Constant  Value=DFES_Cls_DFC_DChrgTCnntMax_C
  DFES_Cls_DFC_BattUNpl_C5 : Constant  Value=DFES_Cls_DFC_CellTempTmt_C
  DFES_Cls_DFC_BattUNpl_C50 : Constant  Value=DFES_Cls_DFC_ChrgOCNpl_C
  DFES_Cls_DFC_BattUNpl_C51 : Constant  Value=DFES_Cls_DFC_DisChOCNpl_C
  DFES_Cls_DFC_BattUNpl_C52 : Constant  Value=DFES_Cls_DFC_BattVoltHiMax_C
  DFES_Cls_DFC_BattUNpl_C53 : Constant  Value=DFES_Cls_DFC_BattVoltLoMin_C
  DFES_Cls_DFC_BattUNpl_C54 : Constant  Value=DFES_Cls_DFC_ThmRnwy_C
  DFES_Cls_DFC_BattUNpl_C55 : Constant  Value=DFES_Cls_DFC_AChrgPortOvrTemp_C
  DFES_Cls_DFC_BattUNpl_C56 : Constant  Value=DFES_Cls_DFC_CurrOffsPlaus_C
  DFES_Cls_DFC_BattUNpl_C57 : Constant  Value=DFES_Cls_DFC_CurrStukPlaus_C
  DFES_Cls_DFC_BattUNpl_C58 : Constant  Value=DFES_Cls_DFC_CurrChrgPlaus_C
  DFES_Cls_DFC_BattUNpl_C59 : Constant  Value=DFES_Cls_DFC_BattUNpl_C
  DFES_Cls_DFC_BattUNpl_C6 : Constant  Value=DFES_Cls_DFC_CellVoltTmt_C
  DFES_Cls_DFC_BattUNpl_C60 : Constant  Value=DFES_Cls_DFC_BattVoltVld_C
  DFES_Cls_DFC_BattUNpl_C61 : Constant  Value=DFES_Cls_DFC_PackUNpl_C
  DFES_Cls_DFC_BattUNpl_C62 : Constant  Value=DFES_Cls_DFC_PackVoltVld_C
  DFES_Cls_DFC_BattUNpl_C63 : Constant  Value=DFES_Cls_DFC_DChrgUNpl_C
  DFES_Cls_DFC_BattUNpl_C64 : Constant  Value=DFES_Cls_DFC_DChrgVoltVld_C
  DFES_Cls_DFC_BattUNpl_C65 : Constant  Value=DFES_Cls_DFC_BoardTempTmt_C
  DFES_Cls_DFC_BattUNpl_C66 : Constant  Value=DFES_Cls_DFC_HvilMax_C
  DFES_Cls_DFC_BattUNpl_C67 : Constant  Value=DFES_Cls_DFC_HvilMin_C
  DFES_Cls_DFC_BattUNpl_C68 : Constant  Value=DFES_Cls_DFC_HvilSig_C
  DFES_Cls_DFC_BattUNpl_C69 : Constant  Value=DFES_Cls_DFC_ChkSumMsg050Err_C
  DFES_Cls_DFC_BattUNpl_C7 : Constant  Value=DFES_Cls_DFC_InCanBusOff_C
  DFES_Cls_DFC_BattUNpl_C70 : Constant  Value=DFES_Cls_DFC_RcMsg050Mis_C
  DFES_Cls_DFC_BattUNpl_C71 : Constant  Value=DFES_Cls_DFC_CrashHwNpl_C
  DFES_Cls_DFC_BattUNpl_C72 : Constant  Value=DFES_Cls_DFC_IsoChkLv1_C
  DFES_Cls_DFC_BattUNpl_C73 : Constant  Value=DFES_Cls_DFC_IsoChkLv2_C
  DFES_Cls_DFC_BattUNpl_C74 : Constant  Value=DFES_Cls_DFC_InsResValdFault_C
  DFES_Cls_DFC_BattUNpl_C75 : Constant  Value=DFES_Cls_DFC_Kl30OutRngErr_C
  DFES_Cls_DFC_BattUNpl_C76 : Constant  Value=DFES_Cls_DFC_Kl30VoltLoErr_C
  DFES_Cls_DFC_BattUNpl_C77 : Constant  Value=DFES_Cls_DFC_Kl30VoltHiErr_C
  DFES_Cls_DFC_BattUNpl_C78 : Constant  Value=DFES_Cls_DFC_EepReadErr_C
  DFES_Cls_DFC_BattUNpl_C79 : Constant  Value=DFES_Cls_DFC_BalStuckMax_C
  DFES_Cls_DFC_BattUNpl_C8 : Constant  Value=DFES_Cls_DFC_VeCanBusOff_C
  DFES_Cls_DFC_BattUNpl_C80 : Constant  Value=DFES_Cls_DFC_BalStuckMin_C
  DFES_Cls_DFC_BattUNpl_C81 : Constant  Value=DFES_Cls_DFC_CSCPwrSpyHiErr_C
  DFES_Cls_DFC_BattUNpl_C82 : Constant  Value=DFES_Cls_DFC_CSCPwrSpyLoErr_C
  DFES_Cls_DFC_BattUNpl_C83 : Constant  Value=DFES_Cls_DFC_CmcBordOTMax_C
  DFES_Cls_DFC_BattUNpl_C84 : Constant  Value=DFES_Cls_DFC_BattTWarnMax_C
  DFES_Cls_DFC_BattUNpl_C85 : Constant  Value=DFES_Cls_DFC_BattTWarnMin_C
  DFES_Cls_DFC_BattUNpl_C86 : Constant  Value=DFES_Cls_DFC_BattTempVldMax_C
  DFES_Cls_DFC_BattUNpl_C87 : Constant  Value=DFES_Cls_DFC_BattTHopMax_C
  DFES_Cls_DFC_BattUNpl_C88 : Constant  Value=DFES_Cls_DFC_CellVoltRngHiErr_C
  DFES_Cls_DFC_BattUNpl_C89 : Constant  Value=DFES_Cls_DFC_CellVoltRngLoErr_C
  DFES_Cls_DFC_BattUNpl_C9 : Constant  Value=DFES_Cls_DFC_Msg2A3Tmt_C
  DFES_Cls_DFC_BattUNpl_C90 : Constant  Value=DFES_Cls_DFC_CellVoltWarnMax_C
  DFES_Cls_DFC_BattUNpl_C91 : Constant  Value=DFES_Cls_DFC_CellVoltWarnMin_C
  DFES_Cls_DFC_BattUNpl_C92 : Constant  Value=DFES_Cls_DFC_CellVoltVldMax_C
  DFES_Cls_DFC_BattUNpl_C93 : Constant  Value=DFES_Cls_DFC_AChrgCurrMish_C
  DFES_Cls_DFC_BattUNpl_C94 : Constant  Value=DFES_Cls_DFC_DChrgCurrMish_C
  DFES_Cls_DFC_BattUNpl_C95 : Constant  Value=DFES_Cls_DFC_DChrgLowTempCurrMish_C
  DFES_Cls_DFC_BattUNpl_C96 : Constant  Value=DFES_Cls_DFC_AChrgVoltMish_C
  DFES_Cls_DFC_BattUNpl_C97 : Constant  Value=DFES_Cls_DFC_DChrgVoltMish_C
  DFES_Cls_DFC_BattUNpl_C98 : Constant  Value=DFES_Cls_DFC_DChrgBattTMin_C
  DFES_Cls_DFC_BattUNpl_C99 : Constant  Value=DFES_Cls_DFC_CC2Chk_C
  DFES_Cls_DFC_BattUNpl_C_zero{,1..252} (253 alike) : Constant  Value=uint8(0)
  Data Type Conversion{,1..8} (9 alike) : DataTypeConversion  OutDataTypeStr=uint8
  FaultLvlCoord : Subsystem
  Logical Operator : Logic  Operator=OR  Inputs=6  AllPortsSameDT=off  OutDataTypeStr=boolean
  Logical Operator1 : Logic  Operator=OR  Inputs=6  AllPortsSameDT=off  OutDataTypeStr=boolean
  Logical Operator2 : Logic  Operator=OR  Inputs=4  AllPortsSameDT=off  OutDataTypeStr=boolean
  Logical Operator{3..6} (4 alike) : Logic  Operator=OR  Inputs=5  AllPortsSameDT=off  OutDataTypeStr=boolean
  Logical Operator7 : Logic  Operator=OR  Inputs=4  AllPortsSameDT=off  OutDataTypeStr=boolean
  MinMax : MinMax  Function=max  Inputs=244
  Relational Operator{1..9} (9 alike) : RelationalOperator  Operator=~=  OutDataTypeStr=boolean  RndMeth=Simplest
  Sum of Elements{,1..8} (9 alike) : Sum  Inputs=+
  DSMR_stFaultRank : Outport
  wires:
  DFC_BattUNpl_1/1 -> DFC_BattUNpl_1_compare/1
  DFC_BattUNpl_1_compare/1 -> DFC_BattUNpl_applied/2
  DFES_Cls_DFC_BattUNpl_C/1 -> DFC_BattUNpl_applied/1
  DFES_Cls_DFC_BattUNpl_C_zero/1 -> DFC_BattUNpl_applied/3
  DFC_CurrRngErr/1 -> DFC_BattUNpl_1/1
  DFC_BattUNpl_2/1 -> DFC_BattUNpl_1_compare1/1
  DFC_BattUNpl_1_compare1/1 -> DFC_BattUNpl_applied1/2
  DFES_Cls_DFC_BattUNpl_C1/1 -> DFC_BattUNpl_applied1/1
  DFES_Cls_DFC_BattUNpl_C_zero1/1 -> DFC_BattUNpl_applied1/3
  DFC_BattVoltRngErr/1 -> DFC_BattUNpl_2/1
  DFC_BattUNpl_3/1 -> DFC_BattUNpl_1_compare2/1
  DFC_BattUNpl_1_compare2/1 -> DFC_BattUNpl_applied2/2
  DFES_Cls_DFC_BattUNpl_C2/1 -> DFC_BattUNpl_applied2/1
  DFES_Cls_DFC_BattUNpl_C_zero2/1 -> DFC_BattUNpl_applied2/3
  DFC_BattHVMsgTmt/1 -> DFC_BattUNpl_3/1
  DFC_BattUNpl_4/1 -> DFC_BattUNpl_1_compare3/1
  DFC_BattUNpl_1_compare3/1 -> DFC_BattUNpl_applied3/2
  DFES_Cls_DFC_BattUNpl_C3/1 -> DFC_BattUNpl_applied3/1
  DFES_Cls_DFC_BattUNpl_C_zero3/1 -> DFC_BattUNpl_applied3/3
  DFC_BusHVMsgTmt/1 -> DFC_BattUNpl_4/1
  DFC_BattUNpl_5/1 -> DFC_BattUNpl_1_compare4/1
  DFC_BattUNpl_1_compare4/1 -> DFC_BattUNpl_applied4/2
  DFES_Cls_DFC_BattUNpl_C4/1 -> DFC_BattUNpl_applied4/1
  DFES_Cls_DFC_BattUNpl_C_zero4/1 -> DFC_BattUNpl_applied4/3
  DFC_638LinCommErr/1 -> DFC_BattUNpl_5/1
  DFC_BattUNpl_6/1 -> DFC_BattUNpl_1_compare5/1
  DFC_BattUNpl_1_compare5/1 -> DFC_BattUNpl_applied5/2
  DFES_Cls_DFC_BattUNpl_C5/1 -> DFC_BattUNpl_applied5/1
  DFES_Cls_DFC_BattUNpl_C_zero5/1 -> DFC_BattUNpl_applied5/3
  DFC_CellTempTmt/1 -> DFC_BattUNpl_6/1
  DFC_BattUNpl_7/1 -> DFC_BattUNpl_1_compare6/1
  DFC_BattUNpl_1_compare6/1 -> DFC_BattUNpl_applied6/2
  DFES_Cls_DFC_BattUNpl_C6/1 -> DFC_BattUNpl_applied6/1
  DFES_Cls_DFC_BattUNpl_C_zero6/1 -> DFC_BattUNpl_applied6/3
  DFC_CellVoltTmt/1 -> DFC_BattUNpl_7/1
  DFC_BattUNpl_8/1 -> DFC_BattUNpl_1_compare7/1
  DFC_BattUNpl_1_compare7/1 -> DFC_BattUNpl_applied7/2
  DFES_Cls_DFC_BattUNpl_C7/1 -> DFC_BattUNpl_applied7/1
  DFES_Cls_DFC_BattUNpl_C_zero7/1 -> DFC_BattUNpl_applied7/3
  DFC_InCanBusOff/1 -> DFC_BattUNpl_8/1
  DFC_BattUNpl_9/1 -> DFC_BattUNpl_1_compare8/1
  DFC_BattUNpl_1_compare8/1 -> DFC_BattUNpl_applied8/2
  DFES_Cls_DFC_BattUNpl_C8/1 -> DFC_BattUNpl_applied8/1
  DFES_Cls_DFC_BattUNpl_C_zero8/1 -> DFC_BattUNpl_applied8/3
  DFC_VeCanBusOff/1 -> DFC_BattUNpl_9/1
  DFC_BattUNpl_10/1 -> DFC_BattUNpl_1_compare9/1
  DFC_BattUNpl_1_compare9/1 -> DFC_BattUNpl_applied9/2
  DFES_Cls_DFC_BattUNpl_C9/1 -> DFC_BattUNpl_applied9/1
  DFES_Cls_DFC_BattUNpl_C_zero9/1 -> DFC_BattUNpl_applied9/3
  DFC_Msg2A3Tmt/1 -> DFC_BattUNpl_10/1
  DFC_BattUNpl_11/1 -> DFC_BattUNpl_1_compare10/1
  DFC_BattUNpl_1_compare10/1 -> DFC_BattUNpl_applied10/2
  DFES_Cls_DFC_BattUNpl_C10/1 -> DFC_BattUNpl_applied10/1
  DFES_Cls_DFC_BattUNpl_C_zero10/1 -> DFC_BattUNpl_applied10/3
  DFC_RcMsg2A3Mis/1 -> DFC_BattUNpl_11/1
  DFC_BattUNpl_12/1 -> DFC_BattUNpl_1_compare11/1
  DFC_BattUNpl_1_compare11/1 -> DFC_BattUNpl_applied11/2
  DFES_Cls_DFC_BattUNpl_C11/1 -> DFC_BattUNpl_applied11/1
  DFES_Cls_DFC_BattUNpl_C_zero11/1 -> DFC_BattUNpl_applied11/3
  DFC_ChkSumMsg2A3Err/1 -> DFC_BattUNpl_12/1
  DFC_BattUNpl_13/1 -> DFC_BattUNpl_1_compare12/1
  DFC_BattUNpl_1_compare12/1 -> DFC_BattUNpl_applied12/2
  DFES_Cls_DFC_BattUNpl_C12/1 -> DFC_BattUNpl_applied12/1
  DFES_Cls_DFC_BattUNpl_C_zero12/1 -> DFC_BattUNpl_applied12/3
  DFC_RcMsg2A5Mis/1 -> DFC_BattUNpl_13/1
  DFC_BattUNpl_14/1 -> DFC_BattUNpl_1_compare13/1
  DFC_BattUNpl_1_compare13/1 -> DFC_BattUNpl_applied13/2
  DFES_Cls_DFC_BattUNpl_C13/1 -> DFC_BattUNpl_applied13/1
  DFES_Cls_DFC_BattUNpl_C_zero13/1 -> DFC_BattUNpl_applied13/3
  DFC_RcMsg2A7Mis/1 -> DFC_BattUNpl_14/1
  DFC_BattUNpl_15/1 -> DFC_BattUNpl_1_compare14/1
  DFC_BattUNpl_1_compare14/1 -> DFC_BattUNpl_applied14/2
  DFES_Cls_DFC_BattUNpl_C14/1 -> DFC_BattUNpl_applied14/1
  DFES_Cls_DFC_BattUNpl_C_zero14/1 -> DFC_BattUNpl_applied14/3
  DFC_CrashNpl/1 -> DFC_BattUNpl_15/1
  DFC_BattUNpl_16/1 -> DFC_BattUNpl_1_compare15/1
  DFC_BattUNpl_1_compare15/1 -> DFC_BattUNpl_applied15/2
  DFES_Cls_DFC_BattUNpl_C15/1 -> DFC_BattUNpl_applied15/1
  DFES_Cls_DFC_BattUNpl_C_zero15/1 -> DFC_BattUNpl_applied15/3
  DFC_FuseNpl/1 -> DFC_BattUNpl_16/1
  DFC_BattUNpl_17/1 -> DFC_BattUNpl_1_compare16/1
  DFC_BattUNpl_1_compare16/1 -> DFC_BattUNpl_applied16/2
  DFES_Cls_DFC_BattUNpl_C16/1 -> DFC_BattUNpl_applied16/1
  DFES_Cls_DFC_BattUNpl_C_zero16/1 -> DFC_BattUNpl_applied16/3
  DFC_Kl30cVoltLoErr/1 -> DFC_BattUNpl_17/1
  DFC_BattUNpl_18/1 -> DFC_BattUNpl_1_compare17/1
  DFC_BattUNpl_1_compare17/1 -> DFC_BattUNpl_applied17/2
  DFES_Cls_DFC_BattUNpl_C17/1 -> DFC_BattUNpl_applied17/1
  DFES_Cls_DFC_BattUNpl_C_zero17/1 -> DFC_BattUNpl_applied17/3
  DFC_PosStuckMax/1 -> DFC_BattUNpl_18/1
  DFC_BattUNpl_19/1 -> DFC_BattUNpl_1_compare18/1
  DFC_BattUNpl_1_compare18/1 -> DFC_BattUNpl_applied18/2
  DFES_Cls_DFC_BattUNpl_C18/1 -> DFC_BattUNpl_applied18/1
  DFES_Cls_DFC_BattUNpl_C_zero18/1 -> DFC_BattUNpl_applied18/3
  DFC_MPosStuckMin/1 -> DFC_BattUNpl_19/1
  DFC_BattUNpl_20/1 -> DFC_BattUNpl_1_compare19/1
  DFC_BattUNpl_1_compare19/1 -> DFC_BattUNpl_applied19/2
  DFES_Cls_DFC_BattUNpl_C19/1 -> DFC_BattUNpl_applied19/1
  DFES_Cls_DFC_BattUNpl_C_zero19/1 -> DFC_BattUNpl_applied19/3
  DFC_MNegStuckMax/1 -> DFC_BattUNpl_20/1
  DFC_BattUNpl_21/1 -> DFC_BattUNpl_1_compare20/1
  DFC_BattUNpl_1_compare20/1 -> DFC_BattUNpl_applied20/2
  DFES_Cls_DFC_BattUNpl_C20/1 -> DFC_BattUNpl_applied20/1
  DFES_Cls_DFC_BattUNpl_C_zero20/1 -> DFC_BattUNpl_applied20/3
  DFC_MNegStuckMin/1 -> DFC_BattUNpl_21/1
  DFC_BattUNpl_22/1 -> DFC_BattUNpl_1_compare21/1
  DFC_BattUNpl_1_compare21/1 -> DFC_BattUNpl_applied21/2
  DFES_Cls_DFC_BattUNpl_C21/1 -> DFC_BattUNpl_applied21/1
  DFES_Cls_DFC_BattUNpl_C_zero21/1 -> DFC_BattUNpl_applied21/3
  DFC_PrStuckMin/1 -> DFC_BattUNpl_22/1
  DFC_BattUNpl_23/1 -> DFC_BattUNpl_1_compare22/1
  DFC_BattUNpl_1_compare22/1 -> DFC_BattUNpl_applied22/2
  DFES_Cls_DFC_BattUNpl_C22/1 -> DFC_BattUNpl_applied22/1
  DFES_Cls_DFC_BattUNpl_C_zero22/1 -> DFC_BattUNpl_applied22/3
  DFC_DChrgPosStuckMax/1 -> DFC_BattUNpl_23/1
  DFC_BattUNpl_24/1 -> DFC_BattUNpl_1_compare23/1
  DFC_BattUNpl_1_compare23/1 -> DFC_BattUNpl_applied23/2
  DFES_Cls_DFC_BattUNpl_C23/1 -> DFC_BattUNpl_applied23/1
  DFES_Cls_DFC_BattUNpl_C_zero23/1 -> DFC_BattUNpl_applied23/3
  DFC_DChrgPosStuckMin/1 -> DFC_BattUNpl_24/1
  DFC_BattUNpl_25/1 -> DFC_BattUNpl_1_compare24/1
  DFC_BattUNpl_1_compare24/1 -> DFC_BattUNpl_applied24/2
  DFES_Cls_DFC_BattUNpl_C24/1 -> DFC_BattUNpl_applied24/1
  DFES_Cls_DFC_BattUNpl_C_zero24/1 -> DFC_BattUNpl_applied24/3
  DFC_DChrgNegStuckMax/1 -> DFC_BattUNpl_25/1
  DFC_BattUNpl_26/1 -> DFC_BattUNpl_1_compare25/1
  DFC_BattUNpl_1_compare25/1 -> DFC_BattUNpl_applied25/2
  DFES_Cls_DFC_BattUNpl_C25/1 -> DFC_BattUNpl_applied25/1
  DFES_Cls_DFC_BattUNpl_C_zero25/1 -> DFC_BattUNpl_applied25/3
  DFC_DChrgNegStuckMin/1 -> DFC_BattUNpl_26/1
  DFC_BattUNpl_27/1 -> DFC_BattUNpl_1_compare26/1
  DFC_BattUNpl_1_compare26/1 -> DFC_BattUNpl_applied26/2
  DFES_Cls_DFC_BattUNpl_C26/1 -> DFC_BattUNpl_applied26/1
  DFES_Cls_DFC_BattUNpl_C_zero26/1 -> DFC_BattUNpl_applied26/3
  DFC_HvPwrUpFail/1 -> DFC_BattUNpl_27/1
  DFC_BattUNpl_28/1 -> DFC_BattUNpl_1_compare27/1
  DFC_BattUNpl_1_compare27/1 -> DFC_BattUNpl_applied27/2
  DFES_Cls_DFC_BattUNpl_C27/1 -> DFC_BattUNpl_applied27/1
  DFES_Cls_DFC_BattUNpl_C_zero27/1 -> DFC_BattUNpl_applied27/3
  DFC_DChrgPwrUpFail/1 -> DFC_BattUNpl_28/1
  DFC_BattUNpl_29/1 -> DFC_BattUNpl_1_compare28/1
  DFC_BattUNpl_1_compare28/1 -> DFC_BattUNpl_applied28/2
  DFES_Cls_DFC_BattUNpl_C28/1 -> DFC_BattUNpl_applied28/1
  DFES_Cls_DFC_BattUNpl_C_zero28/1 -> DFC_BattUNpl_applied28/3
  DFC_BattTAlrmMax/1 -> DFC_BattUNpl_29/1
  DFC_BattUNpl_30/1 -> DFC_BattUNpl_1_compare29/1
  DFC_BattUNpl_1_compare29/1 -> DFC_BattUNpl_applied29/2
  DFES_Cls_DFC_BattUNpl_C29/1 -> DFC_BattUNpl_applied29/1
  DFES_Cls_DFC_BattUNpl_C_zero29/1 -> DFC_BattUNpl_applied29/3
  DFC_BattTFaultMax/1 -> DFC_BattUNpl_30/1
  DFC_BattUNpl_31/1 -> DFC_BattUNpl_1_compare30/1
  DFC_BattUNpl_1_compare30/1 -> DFC_BattUNpl_applied30/2
  DFES_Cls_DFC_BattUNpl_C30/1 -> DFC_BattUNpl_applied30/1
  DFES_Cls_DFC_BattUNpl_C_zero30/1 -> DFC_BattUNpl_applied30/3
  DFC_BattTAlrmMin/1 -> DFC_BattUNpl_31/1
  DFC_BattUNpl_32/1 -> DFC_BattUNpl_1_compare31/1
  DFC_BattUNpl_1_compare31/1 -> DFC_BattUNpl_applied31/2
  DFES_Cls_DFC_BattUNpl_C31/1 -> DFC_BattUNpl_applied31/1
  DFES_Cls_DFC_BattUNpl_C_zero31/1 -> DFC_BattUNpl_applied31/3
  DFC_BattTFaultMin/1 -> DFC_BattUNpl_32/1
  DFC_BattUNpl_33/1 -> DFC_BattUNpl_1_compare32/1
  DFC_BattUNpl_1_compare32/1 -> DFC_BattUNpl_applied32/2
  DFES_Cls_DFC_BattUNpl_C32/1 -> DFC_BattUNpl_applied32/1
  DFES_Cls_DFC_BattUNpl_C_zero32/1 -> DFC_BattUNpl_applied32/3
  DFC_BattTempVldMin/1 -> DFC_BattUNpl_33/1
  DFC_BattUNpl_34/1 -> DFC_BattUNpl_1_compare33/1
  DFC_BattUNpl_1_compare33/1 -> DFC_BattUNpl_applied33/2
  DFES_Cls_DFC_BattUNpl_C33/1 -> DFC_BattUNpl_applied33/1
  DFES_Cls_DFC_BattUNpl_C_zero33/1 -> DFC_BattUNpl_applied33/3
  DFC_BattTCnstMax/1 -> DFC_BattUNpl_34/1
  DFC_BattUNpl_35/1 -> DFC_BattUNpl_1_compare34/1
  DFC_BattUNpl_1_compare34/1 -> DFC_BattUNpl_applied34/2
  DFES_Cls_DFC_BattUNpl_C34/1 -> DFC_BattUNpl_applied34/1
  DFES_Cls_DFC_BattUNpl_C_zero34/1 -> DFC_BattUNpl_applied34/3
  DFC_BattTGradtMax/1 -> DFC_BattUNpl_35/1
  DFC_BattUNpl_36/1 -> DFC_BattUNpl_1_compare35/1
  DFC_BattUNpl_1_compare35/1 -> DFC_BattUNpl_applied35/2
  DFES_Cls_DFC_BattUNpl_C35/1 -> DFC_BattUNpl_applied35/1
  DFES_Cls_DFC_BattUNpl_C_zero35/1 -> DFC_BattUNpl_applied35/3
  DFC_CellVoltAlrmMax/1 -> DFC_BattUNpl_36/1
  DFC_BattUNpl_37/1 -> DFC_BattUNpl_1_compare36/1
  DFC_BattUNpl_1_compare36/1 -> DFC_BattUNpl_applied36/2
  DFES_Cls_DFC_BattUNpl_C36/1 -> DFC_BattUNpl_applied36/1
  DFES_Cls_DFC_BattUNpl_C_zero36/1 -> DFC_BattUNpl_applied36/3
  DFC_CellVoltFaultMax/1 -> DFC_BattUNpl_37/1
  DFC_BattUNpl_38/1 -> DFC_BattUNpl_1_compare37/1
  DFC_BattUNpl_1_compare37/1 -> DFC_BattUNpl_applied37/2
  DFES_Cls_DFC_BattUNpl_C37/1 -> DFC_BattUNpl_applied37/1
  DFES_Cls_DFC_BattUNpl_C_zero37/1 -> DFC_BattUNpl_applied37/3
  DFC_CellVoltFusfMax/1 -> DFC_BattUNpl_38/1
  DFC_BattUNpl_39/1 -> DFC_BattUNpl_1_compare38/1
  DFC_BattUNpl_1_compare38/1 -> DFC_BattUNpl_applied38/2
  DFES_Cls_DFC_BattUNpl_C38/1 -> DFC_BattUNpl_applied38/1
  DFES_Cls_DFC_BattUNpl_C_zero38/1 -> DFC_BattUNpl_applied38/3
  DFC_CellVoltAlrmMin/1 -> DFC_BattUNpl_39/1
  DFC_BattUNpl_40/1 -> DFC_BattUNpl_1_compare39/1
  DFC_BattUNpl_1_compare39/1 -> DFC_BattUNpl_applied39/2
  DFES_Cls_DFC_BattUNpl_C39/1 -> DFC_BattUNpl_applied39/1
  DFES_Cls_DFC_BattUNpl_C_zero39/1 -> DFC_BattUNpl_applied39/3
  DFC_CellVoltFusfMin/1 -> DFC_BattUNpl_40/1
  DFC_BattUNpl_41/1 -> DFC_BattUNpl_1_compare40/1
  DFC_BattUNpl_1_compare40/1 -> DFC_BattUNpl_applied40/2
  DFES_Cls_DFC_BattUNpl_C40/1 -> DFC_BattUNpl_applied40/1
  DFES_Cls_DFC_BattUNpl_C_zero40/1 -> DFC_BattUNpl_applied40/3
  DFC_CellVoltFaultMin/1 -> DFC_BattUNpl_41/1
  DFC_BattUNpl_42/1 -> DFC_BattUNpl_1_compare41/1
  DFC_BattUNpl_1_compare41/1 -> DFC_BattUNpl_applied41/2
  DFES_Cls_DFC_BattUNpl_C41/1 -> DFC_BattUNpl_applied41/1
  DFES_Cls_DFC_BattUNpl_C_zero41/1 -> DFC_BattUNpl_applied41/3
  DFC_CellVoltVldMin/1 -> DFC_BattUNpl_42/1
  DFC_BattUNpl_43/1 -> DFC_BattUNpl_1_compare42/1
  DFC_BattUNpl_1_compare42/1 -> DFC_BattUNpl_applied42/2
  DFES_Cls_DFC_BattUNpl_C42/1 -> DFC_BattUNpl_applied42/1
  DFES_Cls_DFC_BattUNpl_C_zero42/1 -> DFC_BattUNpl_applied42/3
  DFC_CellVoltNpl/1 -> DFC_BattUNpl_43/1
  DFC_BattUNpl_44/1 -> DFC_BattUNpl_1_compare43/1
  DFC_BattUNpl_1_compare43/1 -> DFC_BattUNpl_applied43/2
  DFES_Cls_DFC_BattUNpl_C43/1 -> DFC_BattUNpl_applied43/1
  DFES_Cls_DFC_BattUNpl_C_zero43/1 -> DFC_BattUNpl_applied43/3
  DFC_Msg2E6Tmt/1 -> DFC_BattUNpl_44/1
  DFC_BattUNpl_45/1 -> DFC_BattUNpl_1_compare44/1
  DFC_BattUNpl_1_compare44/1 -> DFC_BattUNpl_applied44/2
  DFES_Cls_DFC_BattUNpl_C44/1 -> DFC_BattUNpl_applied44/1
  DFES_Cls_DFC_BattUNpl_C_zero44/1 -> DFC_BattUNpl_applied44/3
  DFC_RcMsg2E6Mis/1 -> DFC_BattUNpl_45/1
  DFC_BattUNpl_46/1 -> DFC_BattUNpl_1_compare45/1
  DFC_BattUNpl_1_compare45/1 -> DFC_BattUNpl_applied45/2
  DFES_Cls_DFC_BattUNpl_C45/1 -> DFC_BattUNpl_applied45/1
  DFES_Cls_DFC_BattUNpl_C_zero45/1 -> DFC_BattUNpl_applied45/3
  DFC_ChkSumMsg2E6Err/1 -> DFC_BattUNpl_46/1
  DFC_BattUNpl_47/1 -> DFC_BattUNpl_1_compare46/1
  DFC_BattUNpl_1_compare46/1 -> DFC_BattUNpl_applied46/2
  DFES_Cls_DFC_BattUNpl_C46/1 -> DFC_BattUNpl_applied46/1
  DFES_Cls_DFC_BattUNpl_C_zero46/1 -> DFC_BattUNpl_applied46/3
  DFC_RcMsg2E1Mis/1 -> DFC_BattUNpl_47/1
  DFC_BattUNpl_48/1 -> DFC_BattUNpl_1_compare47/1
  DFC_BattUNpl_1_compare47/1 -> DFC_BattUNpl_applied47/2
  DFES_Cls_DFC_BattUNpl_C47/1 -> DFC_BattUNpl_applied47/1
  DFES_Cls_DFC_BattUNpl_C_zero47/1 -> DFC_BattUNpl_applied47/3
  DFC_ChkSumMsg2E1Err/1 -> DFC_BattUNpl_48/1
  DFC_BattUNpl_49/1 -> DFC_BattUNpl_1_compare48/1
  DFC_BattUNpl_1_compare48/1 -> DFC_BattUNpl_applied48/2
  DFES_Cls_DFC_BattUNpl_C48/1 -> DFC_BattUNpl_applied48/1
  DFES_Cls_DFC_BattUNpl_C_zero48/1 -> DFC_BattUNpl_applied48/3
  DFC_DcCanBusOff/1 -> DFC_BattUNpl_49/1
  DFC_BattUNpl_50/1 -> DFC_BattUNpl_1_compare49/1
  DFC_BattUNpl_1_compare49/1 -> DFC_BattUNpl_applied49/2
  DFES_Cls_DFC_BattUNpl_C49/1 -> DFC_BattUNpl_applied49/1
  DFES_Cls_DFC_BattUNpl_C_zero49/1 -> DFC_BattUNpl_applied49/3
  DFC_DChrgTCnntMax/1 -> DFC_BattUNpl_50/1
  DFC_BattUNpl_51/1 -> DFC_BattUNpl_1_compare50/1
  DFC_BattUNpl_1_compare50/1 -> DFC_BattUNpl_applied50/2
  DFES_Cls_DFC_BattUNpl_C50/1 -> DFC_BattUNpl_applied50/1
  DFES_Cls_DFC_BattUNpl_C_zero50/1 -> DFC_BattUNpl_applied50/3
  DFC_ChrgOCNpl/1 -> DFC_BattUNpl_51/1
  DFC_BattUNpl_52/1 -> DFC_BattUNpl_1_compare51/1
  DFC_BattUNpl_1_compare51/1 -> DFC_BattUNpl_applied51/2
  DFES_Cls_DFC_BattUNpl_C51/1 -> DFC_BattUNpl_applied51/1
  DFES_Cls_DFC_BattUNpl_C_zero51/1 -> DFC_BattUNpl_applied51/3
  DFC_DisChOCNpl/1 -> DFC_BattUNpl_52/1
  DFC_BattUNpl_53/1 -> DFC_BattUNpl_1_compare52/1
  DFC_BattUNpl_1_compare52/1 -> DFC_BattUNpl_applied52/2
  DFES_Cls_DFC_BattUNpl_C52/1 -> DFC_BattUNpl_applied52/1
  DFES_Cls_DFC_BattUNpl_C_zero52/1 -> DFC_BattUNpl_applied52/3
  DFC_BattVoltHiMax/1 -> DFC_BattUNpl_53/1
  DFC_BattUNpl_54/1 -> DFC_BattUNpl_1_compare53/1
  DFC_BattUNpl_1_compare53/1 -> DFC_BattUNpl_applied53/2
  DFES_Cls_DFC_BattUNpl_C53/1 -> DFC_BattUNpl_applied53/1
  DFES_Cls_DFC_BattUNpl_C_zero53/1 -> DFC_BattUNpl_applied53/3
  DFC_BattVoltLoMin/1 -> DFC_BattUNpl_54/1
  DFC_BattUNpl_55/1 -> DFC_BattUNpl_1_compare54/1
  DFC_BattUNpl_1_compare54/1 -> DFC_BattUNpl_applied54/2
  DFES_Cls_DFC_BattUNpl_C54/1 -> DFC_BattUNpl_applied54/1
  DFES_Cls_DFC_BattUNpl_C_zero54/1 -> DFC_BattUNpl_applied54/3
  DFC_ThmRnwy/1 -> DFC_BattUNpl_55/1
  DFC_BattUNpl_56/1 -> DFC_BattUNpl_1_compare55/1
  DFC_BattUNpl_1_compare55/1 -> DFC_BattUNpl_applied55/2
  DFES_Cls_DFC_BattUNpl_C55/1 -> DFC_BattUNpl_applied55/1
  DFES_Cls_DFC_BattUNpl_C_zero55/1 -> DFC_BattUNpl_applied55/3
  DFC_AChrgPortOvrTemp/1 -> DFC_BattUNpl_56/1
  DFC_BattUNpl_57/1 -> DFC_BattUNpl_1_compare56/1
  DFC_BattUNpl_1_compare56/1 -> DFC_BattUNpl_applied56/2
  DFES_Cls_DFC_BattUNpl_C56/1 -> DFC_BattUNpl_applied56/1
  DFES_Cls_DFC_BattUNpl_C_zero56/1 -> DFC_BattUNpl_applied56/3
  DFC_CurrOffsPlaus/1 -> DFC_BattUNpl_57/1
  DFC_BattUNpl_58/1 -> DFC_BattUNpl_1_compare57/1
  DFC_BattUNpl_1_compare57/1 -> DFC_BattUNpl_applied57/2
  DFES_Cls_DFC_BattUNpl_C57/1 -> DFC_BattUNpl_applied57/1
  DFES_Cls_DFC_BattUNpl_C_zero57/1 -> DFC_BattUNpl_applied57/3
  DFC_CurrStukPlaus/1 -> DFC_BattUNpl_58/1
  DFC_BattUNpl_59/1 -> DFC_BattUNpl_1_compare58/1
  DFC_BattUNpl_1_compare58/1 -> DFC_BattUNpl_applied58/2
  DFES_Cls_DFC_BattUNpl_C58/1 -> DFC_BattUNpl_applied58/1
  DFES_Cls_DFC_BattUNpl_C_zero58/1 -> DFC_BattUNpl_applied58/3
  DFC_CurrChrgPlaus/1 -> DFC_BattUNpl_59/1
  DFC_BattUNpl_60/1 -> DFC_BattUNpl_1_compare59/1
  DFC_BattUNpl_1_compare59/1 -> DFC_BattUNpl_applied59/2
  DFES_Cls_DFC_BattUNpl_C59/1 -> DFC_BattUNpl_applied59/1
  DFES_Cls_DFC_BattUNpl_C_zero59/1 -> DFC_BattUNpl_applied59/3
  DFC_BattUNpl/1 -> DFC_BattUNpl_60/1
  DFC_BattUNpl_61/1 -> DFC_BattUNpl_1_compare60/1
  DFC_BattUNpl_1_compare60/1 -> DFC_BattUNpl_applied60/2
  DFES_Cls_DFC_BattUNpl_C60/1 -> DFC_BattUNpl_applied60/1
  DFES_Cls_DFC_BattUNpl_C_zero60/1 -> DFC_BattUNpl_applied60/3
  DFC_BattVoltVld/1 -> DFC_BattUNpl_61/1
  DFC_BattUNpl_62/1 -> DFC_BattUNpl_1_compare61/1
  DFC_BattUNpl_1_compare61/1 -> DFC_BattUNpl_applied61/2
  DFES_Cls_DFC_BattUNpl_C61/1 -> DFC_BattUNpl_applied61/1
  DFES_Cls_DFC_BattUNpl_C_zero61/1 -> DFC_BattUNpl_applied61/3
  DFC_PackUNpl/1 -> DFC_BattUNpl_62/1
  DFC_BattUNpl_63/1 -> DFC_BattUNpl_1_compare62/1
  DFC_BattUNpl_1_compare62/1 -> DFC_BattUNpl_applied62/2
  DFES_Cls_DFC_BattUNpl_C62/1 -> DFC_BattUNpl_applied62/1
  DFES_Cls_DFC_BattUNpl_C_zero62/1 -> DFC_BattUNpl_applied62/3
  DFC_PackVoltVld/1 -> DFC_BattUNpl_63/1
  DFC_BattUNpl_64/1 -> DFC_BattUNpl_1_compare63/1
  DFC_BattUNpl_1_compare63/1 -> DFC_BattUNpl_applied63/2
  DFES_Cls_DFC_BattUNpl_C63/1 -> DFC_BattUNpl_applied63/1
  DFES_Cls_DFC_BattUNpl_C_zero63/1 -> DFC_BattUNpl_applied63/3
  DFC_DChrgUNpl/1 -> DFC_BattUNpl_64/1
  DFC_BattUNpl_65/1 -> DFC_BattUNpl_1_compare64/1
  DFC_BattUNpl_1_compare64/1 -> DFC_BattUNpl_applied64/2
  DFES_Cls_DFC_BattUNpl_C64/1 -> DFC_BattUNpl_applied64/1
  DFES_Cls_DFC_BattUNpl_C_zero64/1 -> DFC_BattUNpl_applied64/3
  DFC_DChrgVoltVld/1 -> DFC_BattUNpl_65/1
  DFC_BattUNpl_66/1 -> DFC_BattUNpl_1_compare65/1
  DFC_BattUNpl_1_compare65/1 -> DFC_BattUNpl_applied65/2
  DFES_Cls_DFC_BattUNpl_C65/1 -> DFC_BattUNpl_applied65/1
  DFES_Cls_DFC_BattUNpl_C_zero65/1 -> DFC_BattUNpl_applied65/3
  DFC_BoardTempTmt/1 -> DFC_BattUNpl_66/1
  DFC_BattUNpl_67/1 -> DFC_BattUNpl_1_compare66/1
  DFC_BattUNpl_1_compare66/1 -> DFC_BattUNpl_applied66/2
  DFES_Cls_DFC_BattUNpl_C66/1 -> DFC_BattUNpl_applied66/1
  DFES_Cls_DFC_BattUNpl_C_zero66/1 -> DFC_BattUNpl_applied66/3
  DFC_HvilMax/1 -> DFC_BattUNpl_67/1
  DFC_BattUNpl_68/1 -> DFC_BattUNpl_1_compare67/1
  DFC_BattUNpl_1_compare67/1 -> DFC_BattUNpl_applied67/2
  DFES_Cls_DFC_BattUNpl_C67/1 -> DFC_BattUNpl_applied67/1
  DFES_Cls_DFC_BattUNpl_C_zero67/1 -> DFC_BattUNpl_applied67/3
  DFC_HvilMin/1 -> DFC_BattUNpl_68/1
  DFC_BattUNpl_69/1 -> DFC_BattUNpl_1_compare68/1
  DFC_BattUNpl_1_compare68/1 -> DFC_BattUNpl_applied68/2
  DFES_Cls_DFC_BattUNpl_C68/1 -> DFC_BattUNpl_applied68/1
  DFES_Cls_DFC_BattUNpl_C_zero68/1 -> DFC_BattUNpl_applied68/3
  DFC_HvilSig/1 -> DFC_BattUNpl_69/1
  DFC_BattUNpl_70/1 -> DFC_BattUNpl_1_compare69/1
  DFC_BattUNpl_1_compare69/1 -> DFC_BattUNpl_applied69/2
  DFES_Cls_DFC_BattUNpl_C69/1 -> DFC_BattUNpl_applied69/1
  DFES_Cls_DFC_BattUNpl_C_zero69/1 -> DFC_BattUNpl_applied69/3
  DFC_ChkSumMsg050Err/1 -> DFC_BattUNpl_70/1
  DFC_BattUNpl_71/1 -> DFC_BattUNpl_1_compare70/1
  DFC_BattUNpl_1_compare70/1 -> DFC_BattUNpl_applied70/2
  DFES_Cls_DFC_BattUNpl_C70/1 -> DFC_BattUNpl_applied70/1
  DFES_Cls_DFC_BattUNpl_C_zero70/1 -> DFC_BattUNpl_applied70/3
  DFC_RcMsg050Mis/1 -> DFC_BattUNpl_71/1
  DFC_BattUNpl_72/1 -> DFC_BattUNpl_1_compare71/1
  DFC_BattUNpl_1_compare71/1 -> DFC_BattUNpl_applied71/2
  DFES_Cls_DFC_BattUNpl_C71/1 -> DFC_BattUNpl_applied71/1
  DFES_Cls_DFC_BattUNpl_C_zero71/1 -> DFC_BattUNpl_applied71/3
  DFC_CrashHwNpl/1 -> DFC_BattUNpl_72/1
  DFC_BattUNpl_73/1 -> DFC_BattUNpl_1_compare72/1
  DFC_BattUNpl_1_compare72/1 -> DFC_BattUNpl_applied72/2
  DFES_Cls_DFC_BattUNpl_C72/1 -> DFC_BattUNpl_applied72/1
  DFES_Cls_DFC_BattUNpl_C_zero72/1 -> DFC_BattUNpl_applied72/3
  DFC_IsoChkLv1/1 -> DFC_BattUNpl_73/1
  DFC_BattUNpl_74/1 -> DFC_BattUNpl_1_compare73/1
  DFC_BattUNpl_1_compare73/1 -> DFC_BattUNpl_applied73/2
  DFES_Cls_DFC_BattUNpl_C73/1 -> DFC_BattUNpl_applied73/1
  DFES_Cls_DFC_BattUNpl_C_zero73/1 -> DFC_BattUNpl_applied73/3
  DFC_IsoChkLv2/1 -> DFC_BattUNpl_74/1
  DFC_BattUNpl_75/1 -> DFC_BattUNpl_1_compare74/1
  DFC_BattUNpl_1_compare74/1 -> DFC_BattUNpl_applied74/2
  DFES_Cls_DFC_BattUNpl_C74/1 -> DFC_BattUNpl_applied74/1
  DFES_Cls_DFC_BattUNpl_C_zero74/1 -> DFC_BattUNpl_applied74/3
  DFC_InsResValdFault/1 -> DFC_BattUNpl_75/1
  DFC_BattUNpl_76/1 -> DFC_BattUNpl_1_compare75/1
  DFC_BattUNpl_1_compare75/1 -> DFC_BattUNpl_applied75/2
  DFES_Cls_DFC_BattUNpl_C75/1 -> DFC_BattUNpl_applied75/1
  DFES_Cls_DFC_BattUNpl_C_zero75/1 -> DFC_BattUNpl_applied75/3
  DFC_Kl30OutRngErr/1 -> DFC_BattUNpl_76/1
  DFC_BattUNpl_77/1 -> DFC_BattUNpl_1_compare76/1
  DFC_BattUNpl_1_compare76/1 -> DFC_BattUNpl_applied76/2
  DFES_Cls_DFC_BattUNpl_C76/1 -> DFC_BattUNpl_applied76/1
  DFES_Cls_DFC_BattUNpl_C_zero76/1 -> DFC_BattUNpl_applied76/3
  DFC_Kl30VoltLoErr/1 -> DFC_BattUNpl_77/1
  DFC_BattUNpl_78/1 -> DFC_BattUNpl_1_compare77/1
  DFC_BattUNpl_1_compare77/1 -> DFC_BattUNpl_applied77/2
  DFES_Cls_DFC_BattUNpl_C77/1 -> DFC_BattUNpl_applied77/1
  DFES_Cls_DFC_BattUNpl_C_zero77/1 -> DFC_BattUNpl_applied77/3
  DFC_Kl30VoltHiErr/1 -> DFC_BattUNpl_78/1
  DFC_BattUNpl_79/1 -> DFC_BattUNpl_1_compare78/1
  DFC_BattUNpl_1_compare78/1 -> DFC_BattUNpl_applied78/2
  DFES_Cls_DFC_BattUNpl_C78/1 -> DFC_BattUNpl_applied78/1
  DFES_Cls_DFC_BattUNpl_C_zero78/1 -> DFC_BattUNpl_applied78/3
  DFC_EepReadErr/1 -> DFC_BattUNpl_79/1
  DFC_BattUNpl_80/1 -> DFC_BattUNpl_1_compare79/1
  DFC_BattUNpl_1_compare79/1 -> DFC_BattUNpl_applied79/2
  DFES_Cls_DFC_BattUNpl_C79/1 -> DFC_BattUNpl_applied79/1
  DFES_Cls_DFC_BattUNpl_C_zero79/1 -> DFC_BattUNpl_applied79/3
  DFC_BalStuckMax/1 -> DFC_BattUNpl_80/1
  DFC_BattUNpl_81/1 -> DFC_BattUNpl_1_compare80/1
  DFC_BattUNpl_1_compare80/1 -> DFC_BattUNpl_applied80/2
  DFES_Cls_DFC_BattUNpl_C80/1 -> DFC_BattUNpl_applied80/1
  DFES_Cls_DFC_BattUNpl_C_zero80/1 -> DFC_BattUNpl_applied80/3
  DFC_BalStuckMin/1 -> DFC_BattUNpl_81/1
  DFC_BattUNpl_82/1 -> DFC_BattUNpl_1_compare81/1
  DFC_BattUNpl_1_compare81/1 -> DFC_BattUNpl_applied81/2
  DFES_Cls_DFC_BattUNpl_C81/1 -> DFC_BattUNpl_applied81/1
  DFES_Cls_DFC_BattUNpl_C_zero81/1 -> DFC_BattUNpl_applied81/3
  DFC_CSCPwrSpyHiErr/1 -> DFC_BattUNpl_82/1
  DFC_BattUNpl_83/1 -> DFC_BattUNpl_1_compare82/1
  DFC_BattUNpl_1_compare82/1 -> DFC_BattUNpl_applied82/2
  DFES_Cls_DFC_BattUNpl_C82/1 -> DFC_BattUNpl_applied82/1
  DFES_Cls_DFC_BattUNpl_C_zero82/1 -> DFC_BattUNpl_applied82/3
  DFC_CSCPwrSpyLoErr/1 -> DFC_BattUNpl_83/1
  DFC_BattUNpl_84/1 -> DFC_BattUNpl_1_compare83/1
  DFC_BattUNpl_1_compare83/1 -> DFC_BattUNpl_applied83/2
  DFES_Cls_DFC_BattUNpl_C83/1 -> DFC_BattUNpl_applied83/1
  DFES_Cls_DFC_BattUNpl_C_zero83/1 -> DFC_BattUNpl_applied83/3
  DFC_CmcBordOTMax/1 -> DFC_BattUNpl_84/1
  DFC_BattUNpl_85/1 -> DFC_BattUNpl_1_compare84/1
  DFC_BattUNpl_1_compare84/1 -> DFC_BattUNpl_applied84/2
  DFES_Cls_DFC_BattUNpl_C84/1 -> DFC_BattUNpl_applied84/1
  DFES_Cls_DFC_BattUNpl_C_zero84/1 -> DFC_BattUNpl_applied84/3
  DFC_BattTWarnMax/1 -> DFC_BattUNpl_85/1
  DFC_BattUNpl_86/1 -> DFC_BattUNpl_1_compare85/1
  DFC_BattUNpl_1_compare85/1 -> DFC_BattUNpl_applied85/2
  DFES_Cls_DFC_BattUNpl_C85/1 -> DFC_BattUNpl_applied85/1
  DFES_Cls_DFC_BattUNpl_C_zero85/1 -> DFC_BattUNpl_applied85/3
  DFC_BattTWarnMin/1 -> DFC_BattUNpl_86/1
  DFC_BattUNpl_87/1 -> DFC_BattUNpl_1_compare86/1
  DFC_BattUNpl_1_compare86/1 -> DFC_BattUNpl_applied86/2
  DFES_Cls_DFC_BattUNpl_C86/1 -> DFC_BattUNpl_applied86/1
  DFES_Cls_DFC_BattUNpl_C_zero86/1 -> DFC_BattUNpl_applied86/3
  DFC_BattTempVldMax/1 -> DFC_BattUNpl_87/1
  DFC_BattUNpl_88/1 -> DFC_BattUNpl_1_compare87/1
  DFC_BattUNpl_1_compare87/1 -> DFC_BattUNpl_applied87/2
  DFES_Cls_DFC_BattUNpl_C87/1 -> DFC_BattUNpl_applied87/1
  DFES_Cls_DFC_BattUNpl_C_zero87/1 -> DFC_BattUNpl_applied87/3
  DFC_BattTHopMax/1 -> DFC_BattUNpl_88/1
  DFC_BattUNpl_89/1 -> DFC_BattUNpl_1_compare88/1
  DFC_BattUNpl_1_compare88/1 -> DFC_BattUNpl_applied88/2
  DFES_Cls_DFC_BattUNpl_C88/1 -> DFC_BattUNpl_applied88/1
  DFES_Cls_DFC_BattUNpl_C_zero88/1 -> DFC_BattUNpl_applied88/3
  DFC_CellVoltRngHiErr/1 -> DFC_BattUNpl_89/1
  DFC_BattUNpl_90/1 -> DFC_BattUNpl_1_compare89/1
  DFC_BattUNpl_1_compare89/1 -> DFC_BattUNpl_applied89/2
  DFES_Cls_DFC_BattUNpl_C89/1 -> DFC_BattUNpl_applied89/1
  DFES_Cls_DFC_BattUNpl_C_zero89/1 -> DFC_BattUNpl_applied89/3
  DFC_CellVoltRngLoErr/1 -> DFC_BattUNpl_90/1
  DFC_BattUNpl_91/1 -> DFC_BattUNpl_1_compare90/1
  DFC_BattUNpl_1_compare90/1 -> DFC_BattUNpl_applied90/2
  DFES_Cls_DFC_BattUNpl_C90/1 -> DFC_BattUNpl_applied90/1
  DFES_Cls_DFC_BattUNpl_C_zero90/1 -> DFC_BattUNpl_applied90/3
  DFC_CellVoltWarnMax/1 -> DFC_BattUNpl_91/1
  DFC_BattUNpl_92/1 -> DFC_BattUNpl_1_compare91/1
  DFC_BattUNpl_1_compare91/1 -> DFC_BattUNpl_applied91/2
  DFES_Cls_DFC_BattUNpl_C91/1 -> DFC_BattUNpl_applied91/1
  DFES_Cls_DFC_BattUNpl_C_zero91/1 -> DFC_BattUNpl_applied91/3
  DFC_CellVoltWarnMin/1 -> DFC_BattUNpl_92/1
  DFC_BattUNpl_93/1 -> DFC_BattUNpl_1_compare92/1
  DFC_BattUNpl_1_compare92/1 -> DFC_BattUNpl_applied92/2
  DFES_Cls_DFC_BattUNpl_C92/1 -> DFC_BattUNpl_applied92/1
  DFES_Cls_DFC_BattUNpl_C_zero92/1 -> DFC_BattUNpl_applied92/3
  DFC_CellVoltVldMax/1 -> DFC_BattUNpl_93/1
  DFC_BattUNpl_94/1 -> DFC_BattUNpl_1_compare93/1
  DFC_BattUNpl_1_compare93/1 -> DFC_BattUNpl_applied93/2
  DFES_Cls_DFC_BattUNpl_C93/1 -> DFC_BattUNpl_applied93/1
  DFES_Cls_DFC_BattUNpl_C_zero93/1 -> DFC_BattUNpl_applied93/3
  DFC_AChrgCurrMish/1 -> DFC_BattUNpl_94/1
  DFC_BattUNpl_95/1 -> DFC_BattUNpl_1_compare94/1
  DFC_BattUNpl_1_compare94/1 -> DFC_BattUNpl_applied94/2
  DFES_Cls_DFC_BattUNpl_C94/1 -> DFC_BattUNpl_applied94/1
  DFES_Cls_DFC_BattUNpl_C_zero94/1 -> DFC_BattUNpl_applied94/3
  DFC_DChrgCurrMish/1 -> DFC_BattUNpl_95/1
  DFC_BattUNpl_96/1 -> DFC_BattUNpl_1_compare95/1
  DFC_BattUNpl_1_compare95/1 -> DFC_BattUNpl_applied95/2
  DFES_Cls_DFC_BattUNpl_C95/1 -> DFC_BattUNpl_applied95/1
  DFES_Cls_DFC_BattUNpl_C_zero95/1 -> DFC_BattUNpl_applied95/3
  DFC_DChrgLowTempCurrMish/1 -> DFC_BattUNpl_96/1
  DFC_BattUNpl_97/1 -> DFC_BattUNpl_1_compare96/1
  DFC_BattUNpl_1_compare96/1 -> DFC_BattUNpl_applied96/2
  DFES_Cls_DFC_BattUNpl_C96/1 -> DFC_BattUNpl_applied96/1
  DFES_Cls_DFC_BattUNpl_C_zero96/1 -> DFC_BattUNpl_applied96/3
  DFC_AChrgVoltMish/1 -> DFC_BattUNpl_97/1
  DFC_BattUNpl_98/1 -> DFC_BattUNpl_1_compare97/1
  DFC_BattUNpl_1_compare97/1 -> DFC_BattUNpl_applied97/2
  DFES_Cls_DFC_BattUNpl_C97/1 -> DFC_BattUNpl_applied97/1
  DFES_Cls_DFC_BattUNpl_C_zero97/1 -> DFC_BattUNpl_applied97/3
  DFC_DChrgVoltMish/1 -> DFC_BattUNpl_98/1
  DFC_BattUNpl_99/1 -> DFC_BattUNpl_1_compare98/1
  DFC_BattUNpl_1_compare98/1 -> DFC_BattUNpl_applied98/2
  DFES_Cls_DFC_BattUNpl_C98/1 -> DFC_BattUNpl_applied98/1
  DFES_Cls_DFC_BattUNpl_C_zero98/1 -> DFC_BattUNpl_applied98/3
  DFC_DChrgBattTMin/1 -> DFC_BattUNpl_99/1
  DFC_BattUNpl_100/1 -> DFC_BattUNpl_1_compare99/1
  DFC_BattUNpl_1_compare99/1 -> DFC_BattUNpl_applied99/2
  DFES_Cls_DFC_BattUNpl_C99/1 -> DFC_BattUNpl_applied99/1
  DFES_Cls_DFC_BattUNpl_C_zero99/1 -> DFC_BattUNpl_applied99/3
  DFC_CC2Chk/1 -> DFC_BattUNpl_100/1
  DFC_BattUNpl_101/1 -> DFC_BattUNpl_1_compare100/1
  DFC_BattUNpl_1_compare100/1 -> DFC_BattUNpl_applied100/2
  DFES_Cls_DFC_BattUNpl_C100/1 -> DFC_BattUNpl_applied100/1
  DFES_Cls_DFC_BattUNpl_C_zero100/1 -> DFC_BattUNpl_applied100/3
  DFC_APlusChk/1 -> DFC_BattUNpl_101/1
  DFC_BattUNpl_102/1 -> DFC_BattUNpl_1_compare101/1
  DFC_BattUNpl_1_compare101/1 -> DFC_BattUNpl_applied101/2
  DFES_Cls_DFC_BattUNpl_C101/1 -> DFC_BattUNpl_applied101/1
  DFES_Cls_DFC_BattUNpl_C_zero101/1 -> DFC_BattUNpl_applied101/3
  DFC_DChrgMsgTmt/1 -> DFC_BattUNpl_102/1
  DFC_BattUNpl_103/1 -> DFC_BattUNpl_1_compare102/1
  DFC_BattUNpl_1_compare102/1 -> DFC_BattUNpl_applied102/2
  DFES_Cls_DFC_BattUNpl_C102/1 -> DFC_BattUNpl_applied102/1
  DFES_Cls_DFC_BattUNpl_C_zero102/1 -> DFC_BattUNpl_applied102/3
  DFC_DChrgTNegElecMax/1 -> DFC_BattUNpl_103/1
  DFC_BattUNpl_104/1 -> DFC_BattUNpl_1_compare103/1
  DFC_BattUNpl_1_compare103/1 -> DFC_BattUNpl_applied103/2
  DFES_Cls_DFC_BattUNpl_C103/1 -> DFC_BattUNpl_applied103/1
  DFES_Cls_DFC_BattUNpl_C_zero103/1 -> DFC_BattUNpl_applied103/3
  DFC_DChrgTNegElecMin/1 -> DFC_BattUNpl_104/1
  DFC_BattUNpl_105/1 -> DFC_BattUNpl_1_compare104/1
  DFC_BattUNpl_1_compare104/1 -> DFC_BattUNpl_applied104/2
  DFES_Cls_DFC_BattUNpl_C104/1 -> DFC_BattUNpl_applied104/1
  DFES_Cls_DFC_BattUNpl_C_zero104/1 -> DFC_BattUNpl_applied104/3
  DFC_DChrgTNegElecSig/1 -> DFC_BattUNpl_105/1
  DFC_BattUNpl_106/1 -> DFC_BattUNpl_1_compare105/1
  DFC_BattUNpl_1_compare105/1 -> DFC_BattUNpl_applied105/2
  DFES_Cls_DFC_BattUNpl_C105/1 -> DFC_BattUNpl_applied105/1
  DFES_Cls_DFC_BattUNpl_C_zero105/1 -> DFC_BattUNpl_applied105/3
  DFC_DChrgTPosElecMax/1 -> DFC_BattUNpl_106/1
  DFC_BattUNpl_107/1 -> DFC_BattUNpl_1_compare106/1
  DFC_BattUNpl_1_compare106/1 -> DFC_BattUNpl_applied106/2
  DFES_Cls_DFC_BattUNpl_C106/1 -> DFC_BattUNpl_applied106/1
  DFES_Cls_DFC_BattUNpl_C_zero106/1 -> DFC_BattUNpl_applied106/3
  DFC_DChrgTPosElecMin/1 -> DFC_BattUNpl_107/1
  DFC_BattUNpl_108/1 -> DFC_BattUNpl_1_compare107/1
  DFC_BattUNpl_1_compare107/1 -> DFC_BattUNpl_applied107/2
  DFES_Cls_DFC_BattUNpl_C107/1 -> DFC_BattUNpl_applied107/1
  DFES_Cls_DFC_BattUNpl_C_zero107/1 -> DFC_BattUNpl_applied107/3
  DFC_DChrgTPosElecSig/1 -> DFC_BattUNpl_108/1
  DFC_BattUNpl_109/1 -> DFC_BattUNpl_1_compare108/1
  DFC_BattUNpl_1_compare108/1 -> DFC_BattUNpl_applied108/2
  DFES_Cls_DFC_BattUNpl_C108/1 -> DFC_BattUNpl_applied108/1
  DFES_Cls_DFC_BattUNpl_C_zero108/1 -> DFC_BattUNpl_applied108/3
  DFC_CcuSelfChkErr/1 -> DFC_BattUNpl_109/1
  DFC_BattUNpl_110/1 -> DFC_BattUNpl_1_compare109/1
  DFC_BattUNpl_1_compare109/1 -> DFC_BattUNpl_applied109/2
  DFES_Cls_DFC_BattUNpl_C109/1 -> DFC_BattUNpl_applied109/1
  DFES_Cls_DFC_BattUNpl_C_zero109/1 -> DFC_BattUNpl_applied109/3
  DFC_ChrgOCMin/1 -> DFC_BattUNpl_110/1
  DFC_BattUNpl_111/1 -> DFC_BattUNpl_1_compare110/1
  DFC_BattUNpl_1_compare110/1 -> DFC_BattUNpl_applied110/2
  DFES_Cls_DFC_BattUNpl_C110/1 -> DFC_BattUNpl_applied110/1
  DFES_Cls_DFC_BattUNpl_C_zero110/1 -> DFC_BattUNpl_applied110/3
  DFC_ChrgOCMax/1 -> DFC_BattUNpl_111/1
  DFC_BattUNpl_112/1 -> DFC_BattUNpl_1_compare111/1
  DFC_BattUNpl_1_compare111/1 -> DFC_BattUNpl_applied111/2
  DFES_Cls_DFC_BattUNpl_C111/1 -> DFC_BattUNpl_applied111/1
  DFES_Cls_DFC_BattUNpl_C_zero111/1 -> DFC_BattUNpl_applied111/3
  DFC_DisChOCMin/1 -> DFC_BattUNpl_112/1
  DFC_BattUNpl_113/1 -> DFC_BattUNpl_1_compare112/1
  DFC_BattUNpl_1_compare112/1 -> DFC_BattUNpl_applied112/2
  DFES_Cls_DFC_BattUNpl_C112/1 -> DFC_BattUNpl_applied112/1
  DFES_Cls_DFC_BattUNpl_C_zero112/1 -> DFC_BattUNpl_applied112/3
  DFC_DisChOCMax/1 -> DFC_BattUNpl_113/1
  DFC_BattUNpl_114/1 -> DFC_BattUNpl_1_compare113/1
  DFC_BattUNpl_1_compare113/1 -> DFC_BattUNpl_applied113/2
  DFES_Cls_DFC_BattUNpl_C113/1 -> DFC_BattUNpl_applied113/1
  DFES_Cls_DFC_BattUNpl_C_zero113/1 -> DFC_BattUNpl_applied113/3
  DFC_SocRngLoMax/1 -> DFC_BattUNpl_114/1
  DFC_BattUNpl_115/1 -> DFC_BattUNpl_1_compare114/1
  DFC_BattUNpl_1_compare114/1 -> DFC_BattUNpl_applied114/2
  DFES_Cls_DFC_BattUNpl_C114/1 -> DFC_BattUNpl_applied114/1
  DFES_Cls_DFC_BattUNpl_C_zero114/1 -> DFC_BattUNpl_applied114/3
  DFC_SocRngLoMin/1 -> DFC_BattUNpl_115/1
  DFC_BattUNpl_116/1 -> DFC_BattUNpl_1_compare115/1
  DFC_BattUNpl_1_compare115/1 -> DFC_BattUNpl_applied115/2
  DFES_Cls_DFC_BattUNpl_C115/1 -> DFC_BattUNpl_applied115/1
  DFES_Cls_DFC_BattUNpl_C_zero115/1 -> DFC_BattUNpl_applied115/3
  DFC_SocRngHiMax/1 -> DFC_BattUNpl_116/1
  DFC_BattUNpl_117/1 -> DFC_BattUNpl_1_compare116/1
  DFC_BattUNpl_1_compare116/1 -> DFC_BattUNpl_applied116/2
  DFES_Cls_DFC_BattUNpl_C116/1 -> DFC_BattUNpl_applied116/1
  DFES_Cls_DFC_BattUNpl_C_zero116/1 -> DFC_BattUNpl_applied116/3
  DFC_SocRngHiMin/1 -> DFC_BattUNpl_117/1
  DFC_BattUNpl_118/1 -> DFC_BattUNpl_1_compare117/1
  DFC_BattUNpl_1_compare117/1 -> DFC_BattUNpl_applied117/2
  DFES_Cls_DFC_BattUNpl_C117/1 -> DFC_BattUNpl_applied117/1
  DFES_Cls_DFC_BattUNpl_C_zero117/1 -> DFC_BattUNpl_applied117/3
  DFC_InClntOverTmp/1 -> DFC_BattUNpl_118/1
  DFC_BattUNpl_119/1 -> DFC_BattUNpl_1_compare118/1
  DFC_BattUNpl_1_compare118/1 -> DFC_BattUNpl_applied118/2
  DFES_Cls_DFC_BattUNpl_C118/1 -> DFC_BattUNpl_applied118/1
  DFES_Cls_DFC_BattUNpl_C_zero118/1 -> DFC_BattUNpl_applied118/3
  DFC_OutClntOverTmp/1 -> DFC_BattUNpl_119/1
  DFC_BattUNpl_120/1 -> DFC_BattUNpl_1_compare119/1
  DFC_BattUNpl_1_compare119/1 -> DFC_BattUNpl_applied119/2
  DFES_Cls_DFC_BattUNpl_C119/1 -> DFC_BattUNpl_applied119/1
  DFES_Cls_DFC_BattUNpl_C_zero119/1 -> DFC_BattUNpl_applied119/3
  DFC_ClntDsTElecMax/1 -> DFC_BattUNpl_120/1
  DFC_BattUNpl_121/1 -> DFC_BattUNpl_1_compare120/1
  DFC_BattUNpl_1_compare120/1 -> DFC_BattUNpl_applied120/2
  DFES_Cls_DFC_BattUNpl_C120/1 -> DFC_BattUNpl_applied120/1
  DFES_Cls_DFC_BattUNpl_C_zero120/1 -> DFC_BattUNpl_applied120/3
  DFC_ClntDsTElecMin/1 -> DFC_BattUNpl_121/1
  DFC_BattUNpl_122/1 -> DFC_BattUNpl_1_compare121/1
  DFC_BattUNpl_1_compare121/1 -> DFC_BattUNpl_applied121/2
  DFES_Cls_DFC_BattUNpl_C121/1 -> DFC_BattUNpl_applied121/1
  DFES_Cls_DFC_BattUNpl_C_zero121/1 -> DFC_BattUNpl_applied121/3
  DFC_ClntDsTElecSig/1 -> DFC_BattUNpl_122/1
  DFC_BattUNpl_123/1 -> DFC_BattUNpl_1_compare122/1
  DFC_BattUNpl_1_compare122/1 -> DFC_BattUNpl_applied122/2
  DFES_Cls_DFC_BattUNpl_C122/1 -> DFC_BattUNpl_applied122/1
  DFES_Cls_DFC_BattUNpl_C_zero122/1 -> DFC_BattUNpl_applied122/3
  DFC_ClntUsTElecMax/1 -> DFC_BattUNpl_123/1
  DFC_BattUNpl_124/1 -> DFC_BattUNpl_1_compare123/1
  DFC_BattUNpl_1_compare123/1 -> DFC_BattUNpl_applied123/2
  DFES_Cls_DFC_BattUNpl_C123/1 -> DFC_BattUNpl_applied123/1
  DFES_Cls_DFC_BattUNpl_C_zero123/1 -> DFC_BattUNpl_applied123/3
  DFC_ClntUsTElecMin/1 -> DFC_BattUNpl_124/1
  DFC_BattUNpl_125/1 -> DFC_BattUNpl_1_compare124/1
  DFC_BattUNpl_1_compare124/1 -> DFC_BattUNpl_applied124/2
  DFES_Cls_DFC_BattUNpl_C124/1 -> DFC_BattUNpl_applied124/1
  DFES_Cls_DFC_BattUNpl_C_zero124/1 -> DFC_BattUNpl_applied124/3
  DFC_ClntUsTElecSig/1 -> DFC_BattUNpl_125/1
  DFC_BattUNpl_126/1 -> DFC_BattUNpl_1_compare125/1
  DFC_BattUNpl_1_compare125/1 -> DFC_BattUNpl_applied125/2
  DFES_Cls_DFC_BattUNpl_C125/1 -> DFC_BattUNpl_applied125/1
  DFES_Cls_DFC_BattUNpl_C_zero125/1 -> DFC_BattUNpl_applied125/3
  DFC_CoolPerfPlaus/1 -> DFC_BattUNpl_126/1
  DFC_BattUNpl_127/1 -> DFC_BattUNpl_1_compare126/1
  DFC_BattUNpl_1_compare126/1 -> DFC_BattUNpl_applied126/2
  DFES_Cls_DFC_BattUNpl_C126/1 -> DFC_BattUNpl_applied126/1
  DFES_Cls_DFC_BattUNpl_C_zero126/1 -> DFC_BattUNpl_applied126/3
  DFC_HtgPerfPlaus/1 -> DFC_BattUNpl_127/1
  DFC_BattUNpl_128/1 -> DFC_BattUNpl_1_compare127/1
  DFC_BattUNpl_1_compare127/1 -> DFC_BattUNpl_applied127/2
  DFES_Cls_DFC_BattUNpl_C127/1 -> DFC_BattUNpl_applied127/1
  DFES_Cls_DFC_BattUNpl_C_zero127/1 -> DFC_BattUNpl_applied127/3
  DFC_DChrgFobd/1 -> DFC_BattUNpl_128/1
  DFC_BattUNpl_129/1 -> DFC_BattUNpl_1_compare128/1
  DFC_BattUNpl_1_compare128/1 -> DFC_BattUNpl_applied128/2
  DFES_Cls_DFC_BattUNpl_C128/1 -> DFC_BattUNpl_applied128/1
  DFES_Cls_DFC_BattUNpl_C_zero128/1 -> DFC_BattUNpl_applied128/3
  DFC_DChrgHvOnFail/1 -> DFC_BattUNpl_129/1
  DFC_BattUNpl_130/1 -> DFC_BattUNpl_1_compare129/1
  DFC_BattUNpl_1_compare129/1 -> DFC_BattUNpl_applied129/2
  DFES_Cls_DFC_BattUNpl_C129/1 -> DFC_BattUNpl_applied129/1
  DFES_Cls_DFC_BattUNpl_C_zero129/1 -> DFC_BattUNpl_applied129/3
  DFC_AChgHVOnTmt/1 -> DFC_BattUNpl_130/1
  DFC_BattUNpl_131/1 -> DFC_BattUNpl_1_compare130/1
  DFC_BattUNpl_1_compare130/1 -> DFC_BattUNpl_applied130/2
  DFES_Cls_DFC_BattUNpl_C130/1 -> DFC_BattUNpl_applied130/1
  DFES_Cls_DFC_BattUNpl_C_zero130/1 -> DFC_BattUNpl_applied130/3
  DFC_AChgHVOffTmt/1 -> DFC_BattUNpl_131/1
  DFC_BattUNpl_132/1 -> DFC_BattUNpl_1_compare131/1
  DFC_BattUNpl_1_compare131/1 -> DFC_BattUNpl_applied131/2
  DFES_Cls_DFC_BattUNpl_C131/1 -> DFC_BattUNpl_applied131/1
  DFES_Cls_DFC_BattUNpl_C_zero131/1 -> DFC_BattUNpl_applied131/3
  DFC_AChgS2ClsdTmt/1 -> DFC_BattUNpl_132/1
  DFC_BattUNpl_133/1 -> DFC_BattUNpl_1_compare132/1
  DFC_BattUNpl_1_compare132/1 -> DFC_BattUNpl_applied132/2
  DFES_Cls_DFC_BattUNpl_C132/1 -> DFC_BattUNpl_applied132/1
  DFES_Cls_DFC_BattUNpl_C_zero132/1 -> DFC_BattUNpl_applied132/3
  DFC_DChrgStakeErr/1 -> DFC_BattUNpl_133/1
  DFC_BattUNpl_134/1 -> DFC_BattUNpl_1_compare133/1
  DFC_BattUNpl_1_compare133/1 -> DFC_BattUNpl_applied133/2
  DFES_Cls_DFC_BattUNpl_C133/1 -> DFC_BattUNpl_applied133/1
  DFES_Cls_DFC_BattUNpl_C_zero133/1 -> DFC_BattUNpl_applied133/3
  DFC_DChrgStkVoltErr/1 -> DFC_BattUNpl_134/1
  DFC_BattUNpl_135/1 -> DFC_BattUNpl_1_compare134/1
  DFC_BattUNpl_1_compare134/1 -> DFC_BattUNpl_applied134/2
  DFES_Cls_DFC_BattUNpl_C134/1 -> DFC_BattUNpl_applied134/1
  DFES_Cls_DFC_BattUNpl_C_zero134/1 -> DFC_BattUNpl_applied134/3
  DFC_DChrgStkCurrErr/1 -> DFC_BattUNpl_135/1
  DFC_BattUNpl_136/1 -> DFC_BattUNpl_1_compare135/1
  DFC_BattUNpl_1_compare135/1 -> DFC_BattUNpl_applied135/2
  DFES_Cls_DFC_BattUNpl_C135/1 -> DFC_BattUNpl_applied135/1
  DFES_Cls_DFC_BattUNpl_C_zero135/1 -> DFC_BattUNpl_applied135/3
  DFC_AChgPileRdyTmt/1 -> DFC_BattUNpl_136/1
  DFC_BattUNpl_137/1 -> DFC_BattUNpl_1_compare136/1
  DFC_BattUNpl_1_compare136/1 -> DFC_BattUNpl_applied136/2
  DFES_Cls_DFC_BattUNpl_C136/1 -> DFC_BattUNpl_applied136/1
  DFES_Cls_DFC_BattUNpl_C_zero136/1 -> DFC_BattUNpl_applied136/3
  DFC_DChrgCHMTmt/1 -> DFC_BattUNpl_137/1
  DFC_BattUNpl_138/1 -> DFC_BattUNpl_1_compare137/1
  DFC_BattUNpl_1_compare137/1 -> DFC_BattUNpl_applied137/2
  DFES_Cls_DFC_BattUNpl_C137/1 -> DFC_BattUNpl_applied137/1
  DFES_Cls_DFC_BattUNpl_C_zero137/1 -> DFC_BattUNpl_applied137/3
  DFC_DChrgCRMTmt/1 -> DFC_BattUNpl_138/1
  DFC_BattUNpl_139/1 -> DFC_BattUNpl_1_compare138/1
  DFC_BattUNpl_1_compare138/1 -> DFC_BattUNpl_applied138/2
  DFES_Cls_DFC_BattUNpl_C138/1 -> DFC_BattUNpl_applied138/1
  DFES_Cls_DFC_BattUNpl_C_zero138/1 -> DFC_BattUNpl_applied138/3
  DFC_DChrgCMLTmt/1 -> DFC_BattUNpl_139/1
  DFC_BattUNpl_140/1 -> DFC_BattUNpl_1_compare139/1
  DFC_BattUNpl_1_compare139/1 -> DFC_BattUNpl_applied139/2
  DFES_Cls_DFC_BattUNpl_C139/1 -> DFC_BattUNpl_applied139/1
  DFES_Cls_DFC_BattUNpl_C_zero139/1 -> DFC_BattUNpl_applied139/3
  DFC_DChrgCROTmt/1 -> DFC_BattUNpl_140/1
  DFC_BattUNpl_141/1 -> DFC_BattUNpl_1_compare140/1
  DFC_BattUNpl_1_compare140/1 -> DFC_BattUNpl_applied140/2
  DFES_Cls_DFC_BattUNpl_C140/1 -> DFC_BattUNpl_applied140/1
  DFES_Cls_DFC_BattUNpl_C_zero140/1 -> DFC_BattUNpl_applied140/3
  DFC_DChrgCCSTmt/1 -> DFC_BattUNpl_141/1
  DFC_BattUNpl_142/1 -> DFC_BattUNpl_1_compare141/1
  DFC_BattUNpl_1_compare141/1 -> DFC_BattUNpl_applied141/2
  DFES_Cls_DFC_BattUNpl_C141/1 -> DFC_BattUNpl_applied141/1
  DFES_Cls_DFC_BattUNpl_C_zero141/1 -> DFC_BattUNpl_applied141/3
  DFC_DChrgCSTTmt/1 -> DFC_BattUNpl_142/1
  DFC_BattUNpl_143/1 -> DFC_BattUNpl_1_compare142/1
  DFC_BattUNpl_1_compare142/1 -> DFC_BattUNpl_applied142/2
  DFES_Cls_DFC_BattUNpl_C142/1 -> DFC_BattUNpl_applied142/1
  DFES_Cls_DFC_BattUNpl_C_zero142/1 -> DFC_BattUNpl_applied142/3
  DFC_DChrgCSDTmt/1 -> DFC_BattUNpl_143/1
  DFC_BattUNpl_144/1 -> DFC_BattUNpl_1_compare143/1
  DFC_BattUNpl_1_compare143/1 -> DFC_BattUNpl_applied143/2
  DFES_Cls_DFC_BattUNpl_C143/1 -> DFC_BattUNpl_applied143/1
  DFES_Cls_DFC_BattUNpl_C_zero143/1 -> DFC_BattUNpl_applied143/3
  DFC_DChrgParaChk/1 -> DFC_BattUNpl_144/1
  DFC_BattUNpl_145/1 -> DFC_BattUNpl_1_compare144/1
  DFC_BattUNpl_1_compare144/1 -> DFC_BattUNpl_applied144/2
  DFES_Cls_DFC_BattUNpl_C144/1 -> DFC_BattUNpl_applied144/1
  DFES_Cls_DFC_BattUNpl_C_zero144/1 -> DFC_BattUNpl_applied144/3
  DFC_DChrgCableChk/1 -> DFC_BattUNpl_145/1
  DFC_BattUNpl_146/1 -> DFC_BattUNpl_1_compare145/1
  DFC_BattUNpl_1_compare145/1 -> DFC_BattUNpl_applied145/2
  DFES_Cls_DFC_BattUNpl_C145/1 -> DFC_BattUNpl_applied145/1
  DFES_Cls_DFC_BattUNpl_C_zero145/1 -> DFC_BattUNpl_applied145/3
  DFC_DChrgSLACTOut/1 -> DFC_BattUNpl_146/1
  DFC_BattUNpl_147/1 -> DFC_BattUNpl_1_compare146/1
  DFC_BattUNpl_1_compare146/1 -> DFC_BattUNpl_applied146/2
  DFES_Cls_DFC_BattUNpl_C146/1 -> DFC_BattUNpl_applied146/1
  DFES_Cls_DFC_BattUNpl_C_zero146/1 -> DFC_BattUNpl_applied146/3
  DFC_DChrgCnntErr/1 -> DFC_BattUNpl_147/1
  DFC_BattUNpl_148/1 -> DFC_BattUNpl_1_compare147/1
  DFC_BattUNpl_1_compare147/1 -> DFC_BattUNpl_applied147/2
  DFES_Cls_DFC_BattUNpl_C147/1 -> DFC_BattUNpl_applied147/1
  DFES_Cls_DFC_BattUNpl_C_zero147/1 -> DFC_BattUNpl_applied147/3
  DFC_DChrgLckErr/1 -> DFC_BattUNpl_148/1
  DFC_BattUNpl_149/1 -> DFC_BattUNpl_1_compare148/1
  DFC_BattUNpl_1_compare148/1 -> DFC_BattUNpl_applied148/2
  DFES_Cls_DFC_BattUNpl_C148/1 -> DFC_BattUNpl_applied148/1
  DFES_Cls_DFC_BattUNpl_C_zero148/1 -> DFC_BattUNpl_applied148/3
  DFC_AChrgCnntErr/1 -> DFC_BattUNpl_149/1
  DFC_BattUNpl_150/1 -> DFC_BattUNpl_1_compare149/1
  DFC_BattUNpl_1_compare149/1 -> DFC_BattUNpl_applied149/2
  DFES_Cls_DFC_BattUNpl_C149/1 -> DFC_BattUNpl_applied149/1
  DFES_Cls_DFC_BattUNpl_C_zero149/1 -> DFC_BattUNpl_applied149/3
  DFC_AChgLckTmt/1 -> DFC_BattUNpl_150/1
  DFC_BattUNpl_151/1 -> DFC_BattUNpl_1_compare150/1
  DFC_BattUNpl_1_compare150/1 -> DFC_BattUNpl_applied150/2
  DFES_Cls_DFC_BattUNpl_C150/1 -> DFC_BattUNpl_applied150/1
  DFES_Cls_DFC_BattUNpl_C_zero150/1 -> DFC_BattUNpl_applied150/3
  DFC_AChgRdyPndiTmt/1 -> DFC_BattUNpl_151/1
  DFC_BattUNpl_152/1 -> DFC_BattUNpl_1_compare151/1
  DFC_BattUNpl_1_compare151/1 -> DFC_BattUNpl_applied151/2
  DFES_Cls_DFC_BattUNpl_C151/1 -> DFC_BattUNpl_applied151/1
  DFES_Cls_DFC_BattUNpl_C_zero151/1 -> DFC_BattUNpl_applied151/3
  DFC_AChgRdyTmt/1 -> DFC_BattUNpl_152/1
  DFC_BattUNpl_153/1 -> DFC_BattUNpl_1_compare152/1
  DFC_BattUNpl_1_compare152/1 -> DFC_BattUNpl_applied152/2
  DFES_Cls_DFC_BattUNpl_C152/1 -> DFC_BattUNpl_applied152/1
  DFES_Cls_DFC_BattUNpl_C_zero152/1 -> DFC_BattUNpl_applied152/3
  DFC_AChgingErr/1 -> DFC_BattUNpl_153/1
  DFC_BattUNpl_154/1 -> DFC_BattUNpl_1_compare153/1
  DFC_BattUNpl_1_compare153/1 -> DFC_BattUNpl_applied153/2
  DFES_Cls_DFC_BattUNpl_C153/1 -> DFC_BattUNpl_applied153/1
  DFES_Cls_DFC_BattUNpl_C_zero153/1 -> DFC_BattUNpl_applied153/3
  DFC_AChgUnlckTmt/1 -> DFC_BattUNpl_154/1
  DFC_BattUNpl_155/1 -> DFC_BattUNpl_1_compare154/1
  DFC_BattUNpl_1_compare154/1 -> DFC_BattUNpl_applied154/2
  DFES_Cls_DFC_BattUNpl_C154/1 -> DFC_BattUNpl_applied154/1
  DFES_Cls_DFC_BattUNpl_C_zero154/1 -> DFC_BattUNpl_applied154/3
  DFC_AChgFobd/1 -> DFC_BattUNpl_155/1
  DFC_BattUNpl_156/1 -> DFC_BattUNpl_1_compare155/1
  DFC_BattUNpl_1_compare155/1 -> DFC_BattUNpl_applied155/2
  DFES_Cls_DFC_BattUNpl_C155/1 -> DFC_BattUNpl_applied155/1
  DFES_Cls_DFC_BattUNpl_C_zero155/1 -> DFC_BattUNpl_applied155/3
  DFC_SocValJmp/1 -> DFC_BattUNpl_156/1
  DFC_BattUNpl_applied/1 -> MinMax/1
  DFC_BattUNpl_applied1/1 -> MinMax/2
  DFC_BattUNpl_applied2/1 -> MinMax/3
  DFC_BattUNpl_applied3/1 -> MinMax/4
  DFC_BattUNpl_applied4/1 -> MinMax/5
  DFC_BattUNpl_applied5/1 -> MinMax/6
  DFC_BattUNpl_applied6/1 -> MinMax/7
  DFC_BattUNpl_applied7/1 -> MinMax/8
  DFC_BattUNpl_applied8/1 -> MinMax/9
  DFC_BattUNpl_applied9/1 -> MinMax/10
  DFC_BattUNpl_applied10/1 -> MinMax/11
  DFC_BattUNpl_applied11/1 -> MinMax/12
  DFC_BattUNpl_applied12/1 -> MinMax/13
  DFC_BattUNpl_applied13/1 -> MinMax/14
  DFC_BattUNpl_applied14/1 -> MinMax/15
  DFC_BattUNpl_applied15/1 -> MinMax/16
  DFC_BattUNpl_applied16/1 -> MinMax/17
  DFC_BattUNpl_applied17/1 -> MinMax/18
  DFC_BattUNpl_applied18/1 -> MinMax/19
  DFC_BattUNpl_applied19/1 -> MinMax/20
  DFC_BattUNpl_applied20/1 -> MinMax/21
  DFC_BattUNpl_applied21/1 -> MinMax/22
  DFC_BattUNpl_applied22/1 -> MinMax/23
  DFC_BattUNpl_applied23/1 -> MinMax/24
  DFC_BattUNpl_applied24/1 -> MinMax/25
  DFC_BattUNpl_applied25/1 -> MinMax/26
  DFC_BattUNpl_applied26/1 -> MinMax/27
  DFC_BattUNpl_applied27/1 -> MinMax/28
  DFC_BattUNpl_applied28/1 -> MinMax/29
  DFC_BattUNpl_applied29/1 -> MinMax/30
  DFC_BattUNpl_applied30/1 -> MinMax/31
  DFC_BattUNpl_applied31/1 -> MinMax/32
  DFC_BattUNpl_applied32/1 -> MinMax/33
  DFC_BattUNpl_applied33/1 -> MinMax/34
  DFC_BattUNpl_applied34/1 -> MinMax/35
  DFC_BattUNpl_applied35/1 -> MinMax/36
  DFC_BattUNpl_applied36/1 -> MinMax/37
  DFC_BattUNpl_applied37/1 -> MinMax/38
  DFC_BattUNpl_applied38/1 -> MinMax/39
  DFC_BattUNpl_applied39/1 -> MinMax/40
  DFC_BattUNpl_applied40/1 -> MinMax/41
  DFC_BattUNpl_applied41/1 -> MinMax/42
  DFC_BattUNpl_applied42/1 -> MinMax/43
  DFC_BattUNpl_applied43/1 -> MinMax/44
  DFC_BattUNpl_applied44/1 -> MinMax/45
  DFC_BattUNpl_applied45/1 -> MinMax/46
  DFC_BattUNpl_applied46/1 -> MinMax/47
  DFC_BattUNpl_applied47/1 -> MinMax/48
  DFC_BattUNpl_applied48/1 -> MinMax/49
  DFC_BattUNpl_applied49/1 -> MinMax/50
  DFC_BattUNpl_applied50/1 -> MinMax/51
  DFC_BattUNpl_applied51/1 -> MinMax/52
  DFC_BattUNpl_applied52/1 -> MinMax/53
  DFC_BattUNpl_applied53/1 -> MinMax/54
  DFC_BattUNpl_applied54/1 -> MinMax/55
  DFC_BattUNpl_applied55/1 -> MinMax/56
  DFC_BattUNpl_applied56/1 -> MinMax/57
  DFC_BattUNpl_applied57/1 -> MinMax/58
  DFC_BattUNpl_applied58/1 -> MinMax/59
  DFC_BattUNpl_applied59/1 -> MinMax/60
  DFC_BattUNpl_applied60/1 -> MinMax/61
  DFC_BattUNpl_applied61/1 -> MinMax/62
  DFC_BattUNpl_applied62/1 -> MinMax/63
  DFC_BattUNpl_applied63/1 -> MinMax/64
  DFC_BattUNpl_applied64/1 -> MinMax/65
  DFC_BattUNpl_applied65/1 -> MinMax/66
  DFC_BattUNpl_applied66/1 -> MinMax/67
  DFC_BattUNpl_applied67/1 -> MinMax/68
  DFC_BattUNpl_applied68/1 -> MinMax/69
  DFC_BattUNpl_applied69/1 -> MinMax/70
  DFC_BattUNpl_applied70/1 -> MinMax/71
  DFC_BattUNpl_applied71/1 -> MinMax/72
  DFC_BattUNpl_applied72/1 -> MinMax/73
  DFC_BattUNpl_applied73/1 -> MinMax/74
  DFC_BattUNpl_applied74/1 -> MinMax/75
  DFC_BattUNpl_applied75/1 -> MinMax/76
  DFC_BattUNpl_applied76/1 -> MinMax/77
  DFC_BattUNpl_applied77/1 -> MinMax/78
  DFC_BattUNpl_applied78/1 -> MinMax/79
  DFC_BattUNpl_applied79/1 -> MinMax/80
  DFC_BattUNpl_applied80/1 -> MinMax/81
  DFC_BattUNpl_applied81/1 -> MinMax/82
  DFC_BattUNpl_applied82/1 -> MinMax/83
  DFC_BattUNpl_applied83/1 -> MinMax/84
  DFC_BattUNpl_applied84/1 -> MinMax/85
  DFC_BattUNpl_applied85/1 -> MinMax/86
  DFC_BattUNpl_applied86/1 -> MinMax/87
  DFC_BattUNpl_applied87/1 -> MinMax/88
  DFC_BattUNpl_applied88/1 -> MinMax/89
  DFC_BattUNpl_applied89/1 -> MinMax/90
  DFC_BattUNpl_applied90/1 -> MinMax/91
  DFC_BattUNpl_applied91/1 -> MinMax/92
  DFC_BattUNpl_applied92/1 -> MinMax/93
  DFC_BattUNpl_applied93/1 -> MinMax/94
  DFC_BattUNpl_applied94/1 -> MinMax/95
  DFC_BattUNpl_applied95/1 -> MinMax/96
  DFC_BattUNpl_applied96/1 -> MinMax/97
  DFC_BattUNpl_applied97/1 -> MinMax/98
  DFC_BattUNpl_applied98/1 -> MinMax/99
  DFC_BattUNpl_applied99/1 -> MinMax/100
  DFC_BattUNpl_applied100/1 -> MinMax/101
  DFC_BattUNpl_applied101/1 -> MinMax/102
  DFC_BattUNpl_applied102/1 -> MinMax/103
  DFC_BattUNpl_applied103/1 -> MinMax/104
  DFC_BattUNpl_applied104/1 -> MinMax/105
  DFC_BattUNpl_applied105/1 -> MinMax/106
  DFC_BattUNpl_applied106/1 -> MinMax/107
  DFC_BattUNpl_applied107/1 -> MinMax/108
  DFC_BattUNpl_applied108/1 -> MinMax/109
  DFC_BattUNpl_applied109/1 -> MinMax/110
  DFC_BattUNpl_applied110/1 -> MinMax/111
  DFC_BattUNpl_applied111/1 -> MinMax/112
  DFC_BattUNpl_applied112/1 -> MinMax/113
  DFC_BattUNpl_applied113/1 -> MinMax/114
  DFC_BattUNpl_applied114/1 -> MinMax/115
  DFC_BattUNpl_applied115/1 -> MinMax/116
  DFC_BattUNpl_applied116/1 -> MinMax/117
  DFC_BattUNpl_applied117/1 -> MinMax/118
  DFC_BattUNpl_applied118/1 -> MinMax/119
  DFC_BattUNpl_applied119/1 -> MinMax/120
  DFC_BattUNpl_applied120/1 -> MinMax/121
  DFC_BattUNpl_applied121/1 -> MinMax/122
  DFC_BattUNpl_applied122/1 -> MinMax/123
  DFC_BattUNpl_applied123/1 -> MinMax/124
  DFC_BattUNpl_applied124/1 -> MinMax/125
  DFC_BattUNpl_applied125/1 -> MinMax/126
  DFC_BattUNpl_applied126/1 -> MinMax/127
  DFC_BattUNpl_applied127/1 -> MinMax/128
  DFC_BattUNpl_applied128/1 -> MinMax/129
  DFC_BattUNpl_applied129/1 -> MinMax/130
  DFC_BattUNpl_applied130/1 -> MinMax/131
  DFC_BattUNpl_applied131/1 -> MinMax/132
  DFC_BattUNpl_applied132/1 -> MinMax/133
  DFC_BattUNpl_applied133/1 -> MinMax/134
  DFC_BattUNpl_applied134/1 -> MinMax/135
  DFC_BattUNpl_applied135/1 -> MinMax/136
  DFC_BattUNpl_applied136/1 -> MinMax/137
  DFC_BattUNpl_applied137/1 -> MinMax/138
  DFC_BattUNpl_applied138/1 -> MinMax/139
  DFC_BattUNpl_applied139/1 -> MinMax/140
  DFC_BattUNpl_applied140/1 -> MinMax/141
  DFC_BattUNpl_applied141/1 -> MinMax/142
  DFC_BattUNpl_applied142/1 -> MinMax/143
  DFC_BattUNpl_applied143/1 -> MinMax/144
  DFC_BattUNpl_applied144/1 -> MinMax/145
  DFC_BattUNpl_applied145/1 -> MinMax/146
  DFC_BattUNpl_applied146/1 -> MinMax/147
  DFC_BattUNpl_applied147/1 -> MinMax/148
  DFC_BattUNpl_applied148/1 -> MinMax/149
  DFC_BattUNpl_applied149/1 -> MinMax/150
  DFC_BattUNpl_applied150/1 -> MinMax/151
  DFC_BattUNpl_applied151/1 -> MinMax/152
  DFC_BattUNpl_applied152/1 -> MinMax/153
  DFC_BattUNpl_applied153/1 -> MinMax/154
  DFC_BattUNpl_applied154/1 -> MinMax/155
  DFC_BattUNpl_applied155/1 -> MinMax/156
  MinMax/1 -> FaultLvlCoord/1(DSMR_stFaultRankRaw)
  FaultLvlCoord/1(DSMR_stFaultRank) -> DSMR_stFaultRank/1
  DFC_BattUNpl_157/1 -> DFC_BattUNpl_1_compare156/1
  DFC_BattUNpl_1_compare156/1 -> DFC_BattUNpl_applied156/2
  DFES_Cls_DFC_BattUNpl_C156/1 -> DFC_BattUNpl_applied156/1
  DFES_Cls_DFC_BattUNpl_C_zero156/1 -> DFC_BattUNpl_applied156/3
  DFC_ChrgCmuLost/1 -> DFC_BattUNpl_157/1
  DFC_BattUNpl_applied156/1 -> MinMax/157
  DFC_BattUNpl_158/1 -> DFC_BattUNpl_1_compare157/1
  DFC_BattUNpl_1_compare157/1 -> DFC_BattUNpl_applied157/2
  DFES_Cls_DFC_BattUNpl_C157/1 -> DFC_BattUNpl_applied157/1
  DFES_Cls_DFC_BattUNpl_C_zero157/1 -> DFC_BattUNpl_applied157/3
  DFC_DisChrgCmuLost/1 -> DFC_BattUNpl_158/1
  DFC_BattUNpl_applied157/1 -> MinMax/158
  DFC_BattUNpl_159/1 -> DFC_BattUNpl_1_compare158/1
  DFC_BattUNpl_1_compare158/1 -> DFC_BattUNpl_applied158/2
  DFES_Cls_DFC_BattUNpl_C158/1 -> DFC_BattUNpl_applied158/1
  DFES_Cls_DFC_BattUNpl_C_zero158/1 -> DFC_BattUNpl_applied158/3
  DFC_Msg130Tmt/1 -> DFC_BattUNpl_159/1
  DFC_BattUNpl_applied158/1 -> MinMax/159
  DFC_BattUNpl_160/1 -> DFC_BattUNpl_1_compare159/1
  DFC_BattUNpl_1_compare159/1 -> DFC_BattUNpl_applied159/2
  DFES_Cls_DFC_BattUNpl_C159/1 -> DFC_BattUNpl_applied159/1
  DFES_Cls_DFC_BattUNpl_C_zero159/1 -> DFC_BattUNpl_applied159/3
  DFC_Msg2E1Tmt/1 -> DFC_BattUNpl_160/1
  DFC_BattUNpl_applied159/1 -> MinMax/160
  DFC_BattUNpl_161/1 -> DFC_BattUNpl_1_compare160/1
  DFC_BattUNpl_1_compare160/1 -> DFC_BattUNpl_applied160/2
  DFES_Cls_DFC_BattUNpl_C160/1 -> DFC_BattUNpl_applied160/1
  DFES_Cls_DFC_BattUNpl_C_zero160/1 -> DFC_BattUNpl_applied160/3
  DFC_BattUNpl_162/1 -> DFC_BattUNpl_1_compare161/1
  DFC_BattUNpl_1_compare161/1 -> DFC_BattUNpl_applied161/2
  DFES_Cls_DFC_BattUNpl_C161/1 -> DFC_BattUNpl_applied161/1
  DFES_Cls_DFC_BattUNpl_C_zero161/1 -> DFC_BattUNpl_applied161/3
  DFC_BattUNpl_163/1 -> DFC_BattUNpl_1_compare162/1
  DFC_BattUNpl_1_compare162/1 -> DFC_BattUNpl_applied162/2
  DFES_Cls_DFC_BattUNpl_C162/1 -> DFC_BattUNpl_applied162/1
  DFES_Cls_DFC_BattUNpl_C_zero162/1 -> DFC_BattUNpl_applied162/3
  DFC_BattUNpl_164/1 -> DFC_BattUNpl_1_compare163/1
  DFC_BattUNpl_1_compare163/1 -> DFC_BattUNpl_applied163/2
  DFES_Cls_DFC_BattUNpl_C163/1 -> DFC_BattUNpl_applied163/1
  DFES_Cls_DFC_BattUNpl_C_zero163/1 -> DFC_BattUNpl_applied163/3
  DFC_BattUNpl_165/1 -> DFC_BattUNpl_1_compare164/1
  DFC_BattUNpl_1_compare164/1 -> DFC_BattUNpl_applied164/2
  DFES_Cls_DFC_BattUNpl_C164/1 -> DFC_BattUNpl_applied164/1
  DFES_Cls_DFC_BattUNpl_C_zero164/1 -> DFC_BattUNpl_applied164/3
  DFC_BattUNpl_166/1 -> DFC_BattUNpl_1_compare165/1
  DFC_BattUNpl_1_compare165/1 -> DFC_BattUNpl_applied165/2
  DFES_Cls_DFC_BattUNpl_C165/1 -> DFC_BattUNpl_applied165/1
  DFES_Cls_DFC_BattUNpl_C_zero165/1 -> DFC_BattUNpl_applied165/3
  DFC_Msg2EBTmt/1 -> DFC_BattUNpl_161/1
  DFC_MsgCABTmt/1 -> DFC_BattUNpl_162/1
  DFC_BattUNpl_applied160/1 -> MinMax/161
  DFC_BattUNpl_applied161/1 -> MinMax/162
  DFC_BattUNpl_applied162/1 -> MinMax/163
  DFC_BattUNpl_applied163/1 -> MinMax/164
  DFC_BattUNpl_applied164/1 -> MinMax/165
  DFC_BattUNpl_applied165/1 -> MinMax/166
  DFC_Msg0B5Tmt/1 -> DFC_BattUNpl_163/1
  DFC_ObcTmt/1 -> DFC_BattUNpl_164/1
  DFC_VcuTmt/1 -> DFC_BattUNpl_165/1
  DFC_Msg2A7Tmt/1 -> DFC_BattUNpl_166/1
  DFC_BattUNpl_167/1 -> DFC_BattUNpl_1_compare166/1
  DFC_BattUNpl_1_compare166/1 -> DFC_BattUNpl_applied166/2
  DFES_Cls_DFC_BattUNpl_C_zero166/1 -> DFC_BattUNpl_applied166/3
  DFC_BattUNpl_168/1 -> DFC_BattUNpl_1_compare167/1
  DFC_BattUNpl_1_compare167/1 -> DFC_BattUNpl_applied167/2
  DFES_Cls_DFC_BattUNpl_C167/1 -> DFC_BattUNpl_applied167/1
  DFES_Cls_DFC_BattUNpl_C_zero167/1 -> DFC_BattUNpl_applied167/3
  DFC_BattUNpl_169/1 -> DFC_BattUNpl_1_compare168/1
  DFC_BattUNpl_1_compare168/1 -> DFC_BattUNpl_applied168/2
  DFES_Cls_DFC_BattUNpl_C168/1 -> DFC_BattUNpl_applied168/1
  DFES_Cls_DFC_BattUNpl_C_zero168/1 -> DFC_BattUNpl_applied168/3
  DFC_BattUNpl_170/1 -> DFC_BattUNpl_1_compare169/1
  DFC_BattUNpl_1_compare169/1 -> DFC_BattUNpl_applied169/2
  DFES_Cls_DFC_BattUNpl_C169/1 -> DFC_BattUNpl_applied169/1
  DFES_Cls_DFC_BattUNpl_C_zero169/1 -> DFC_BattUNpl_applied169/3
  DFC_BattUNpl_171/1 -> DFC_BattUNpl_1_compare170/1
  DFC_BattUNpl_1_compare170/1 -> DFC_BattUNpl_applied170/2
  DFES_Cls_DFC_BattUNpl_C_zero170/1 -> DFC_BattUNpl_applied170/3
  DFC_BattUNpl_172/1 -> DFC_BattUNpl_1_compare171/1
  DFC_BattUNpl_1_compare171/1 -> DFC_BattUNpl_applied171/2
  DFES_Cls_DFC_BattUNpl_C171/1 -> DFC_BattUNpl_applied171/1
  DFES_Cls_DFC_BattUNpl_C_zero171/1 -> DFC_BattUNpl_applied171/3
  DFC_BattUNpl_173/1 -> DFC_BattUNpl_1_compare172/1
  DFC_BattUNpl_1_compare172/1 -> DFC_BattUNpl_applied172/2
  DFES_Cls_DFC_BattUNpl_C172/1 -> DFC_BattUNpl_applied172/1
  DFES_Cls_DFC_BattUNpl_C_zero172/1 -> DFC_BattUNpl_applied172/3
  DFC_BattUNpl_174/1 -> DFC_BattUNpl_1_compare173/1
  DFC_BattUNpl_1_compare173/1 -> DFC_BattUNpl_applied173/2
  DFES_Cls_DFC_BattUNpl_C173/1 -> DFC_BattUNpl_applied173/1
  DFES_Cls_DFC_BattUNpl_C_zero173/1 -> DFC_BattUNpl_applied173/3
  DFC_BattUNpl_applied170/1 -> MinMax/171
  DFC_BattUNpl_applied171/1 -> MinMax/172
  DFC_BattUNpl_applied173/1 -> MinMax/174
  DFC_BattUNpl_applied166/1 -> MinMax/167
  DFC_BattUNpl_applied167/1 -> MinMax/168
  DFC_BattUNpl_applied172/1 -> MinMax/173
  DFC_BattUNpl_applied168/1 -> MinMax/169
  DFC_BattUNpl_applied169/1 -> MinMax/170
  DFES_Cls_DFC_BattUNpl_C170/1 -> DFC_BattUNpl_applied170/1
  DFES_Cls_DFC_BattUNpl_C166/1 -> DFC_BattUNpl_applied166/1
  DFC_BattUNpl_175/1 -> DFC_BattUNpl_1_compare174/1
  DFC_BattUNpl_1_compare174/1 -> DFC_BattUNpl_applied174/2
  DFES_Cls_DFC_BattUNpl_C174/1 -> DFC_BattUNpl_applied174/1
  DFES_Cls_DFC_BattUNpl_C_zero174/1 -> DFC_BattUNpl_applied174/3
  DFC_BattUNpl_176/1 -> DFC_BattUNpl_1_compare175/1
  DFC_BattUNpl_1_compare175/1 -> DFC_BattUNpl_applied175/2
  DFES_Cls_DFC_BattUNpl_C175/1 -> DFC_BattUNpl_applied175/1
  DFES_Cls_DFC_BattUNpl_C_zero175/1 -> DFC_BattUNpl_applied175/3
  DFC_BattUNpl_177/1 -> DFC_BattUNpl_1_compare176/1
  DFC_BattUNpl_1_compare176/1 -> DFC_BattUNpl_applied176/2
  DFES_Cls_DFC_BattUNpl_C_zero176/1 -> DFC_BattUNpl_applied176/3
  DFC_BattUNpl_178/1 -> DFC_BattUNpl_1_compare177/1
  DFC_BattUNpl_1_compare177/1 -> DFC_BattUNpl_applied177/2
  DFES_Cls_DFC_BattUNpl_C177/1 -> DFC_BattUNpl_applied177/1
  DFES_Cls_DFC_BattUNpl_C_zero177/1 -> DFC_BattUNpl_applied177/3
  DFC_BattUNpl_179/1 -> DFC_BattUNpl_1_compare178/1
  DFC_BattUNpl_1_compare178/1 -> DFC_BattUNpl_applied178/2
  DFES_Cls_DFC_BattUNpl_C178/1 -> DFC_BattUNpl_applied178/1
  DFES_Cls_DFC_BattUNpl_C_zero178/1 -> DFC_BattUNpl_applied178/3
  DFC_BattUNpl_180/1 -> DFC_BattUNpl_1_compare179/1
  DFC_BattUNpl_1_compare179/1 -> DFC_BattUNpl_applied179/2
  DFES_Cls_DFC_BattUNpl_C179/1 -> DFC_BattUNpl_applied179/1
  DFES_Cls_DFC_BattUNpl_C_zero179/1 -> DFC_BattUNpl_applied179/3
  DFES_Cls_DFC_BattUNpl_C176/1 -> DFC_BattUNpl_applied176/1
  DFC_BattUNpl_applied177/1 -> MinMax/178
  DFC_BattUNpl_applied176/1 -> MinMax/177
  DFC_BattUNpl_applied178/1 -> MinMax/179
  DFC_BattUNpl_applied179/1 -> MinMax/180
  DFC_BattUNpl_applied174/1 -> MinMax/175
  DFC_BattUNpl_applied175/1 -> MinMax/176
  DFC_Msg2A5Tmt/1 -> DFC_BattUNpl_167/1
  DFC_Msg2ADTmt/1 -> DFC_BattUNpl_168/1
  DFC_Msg2BBTmt/1 -> DFC_BattUNpl_169/1
  DFC_Msg2DFTmt/1 -> DFC_BattUNpl_170/1
  DFC_BattCurrMismatchErr/1 -> DFC_BattUNpl_180/1
  DFC_CABErr/1 -> DFC_BattUNpl_179/1
  DFC_HwCurrElecSCP/1 -> DFC_BattUNpl_178/1
  DFC_HwCurrElecSCG/1 -> DFC_BattUNpl_177/1
  DFC_Msg17DTmt/1 -> DFC_BattUNpl_176/1
  DFC_Msg28CTmt/1 -> DFC_BattUNpl_175/1
  DFC_Msg37FTmt/1 -> DFC_BattUNpl_174/1
  DFC_Msg3AATmt/1 -> DFC_BattUNpl_171/1
  DFC_Msg050Tmt/1 -> DFC_BattUNpl_172/1
  DFC_Msg2F1Tmt/1 -> DFC_BattUNpl_173/1
  DFC_BattUNpl_181/1 -> DFC_BattUNpl_1_compare180/1
  DFC_BattUNpl_1_compare180/1 -> DFC_BattUNpl_applied180/2
  DFES_Cls_DFC_BattUNpl_C_zero180/1 -> DFC_BattUNpl_applied180/3
  DFC_BattUNpl_applied180/1 -> MinMax/181
  DFC_Msg195Tmt/1 -> DFC_BattUNpl_181/1
  DFES_Cls_DFC_BattUNpl_C180/1 -> DFC_BattUNpl_applied180/1
  Relational Operator1/1 -> DFC_BattUNpl_applied181/2
  DFES_Cls_DFC_BattUNpl_C_zero181/1 -> DFC_BattUNpl_applied181/3
  DFES_Cls_DFC_BattUNpl_C181/1 -> DFC_BattUNpl_applied181/1
  DFC_BattUNpl_applied181/1 -> MinMax/182
  DFES_Cls_DFC_BattUNpl_C_zero182/1 -> DFC_BattUNpl_applied182/3
  DFES_Cls_DFC_BattUNpl_C182/1 -> DFC_BattUNpl_applied182/1
  Relational Operator3/1 -> DFC_BattUNpl_applied183/2
  DFES_Cls_DFC_BattUNpl_C_zero183/1 -> DFC_BattUNpl_applied183/3
  DFES_Cls_DFC_BattUNpl_C183/1 -> DFC_BattUNpl_applied183/1
  Relational Operator4/1 -> DFC_BattUNpl_applied184/2
  DFES_Cls_DFC_BattUNpl_C_zero184/1 -> DFC_BattUNpl_applied184/3
  DFES_Cls_DFC_BattUNpl_C184/1 -> DFC_BattUNpl_applied184/1
  Relational Operator5/1 -> DFC_BattUNpl_applied185/2
  DFES_Cls_DFC_BattUNpl_C_zero185/1 -> DFC_BattUNpl_applied185/3
  DFES_Cls_DFC_BattUNpl_C185/1 -> DFC_BattUNpl_applied185/1
  Relational Operator6/1 -> DFC_BattUNpl_applied186/2
  DFES_Cls_DFC_BattUNpl_C_zero186/1 -> DFC_BattUNpl_applied186/3
  DFES_Cls_DFC_BattUNpl_C186/1 -> DFC_BattUNpl_applied186/1
  Relational Operator7/1 -> DFC_BattUNpl_applied187/2
  DFES_Cls_DFC_BattUNpl_C_zero187/1 -> DFC_BattUNpl_applied187/3
  DFES_Cls_DFC_BattUNpl_C187/1 -> DFC_BattUNpl_applied187/1
  Relational Operator8/1 -> DFC_BattUNpl_applied188/2
  DFES_Cls_DFC_BattUNpl_C_zero188/1 -> DFC_BattUNpl_applied188/3
  DFES_Cls_DFC_BattUNpl_C188/1 -> DFC_BattUNpl_applied188/1
  Relational Operator9/1 -> DFC_BattUNpl_applied189/2
  DFES_Cls_DFC_BattUNpl_C_zero189/1 -> DFC_BattUNpl_applied189/3
  DFES_Cls_DFC_BattUNpl_C189/1 -> DFC_BattUNpl_applied189/1
  DFC_BattUNpl_applied182/1 -> MinMax/183
  DFC_BattUNpl_applied183/1 -> MinMax/184
  DFC_BattUNpl_applied184/1 -> MinMax/185
  DFC_BattUNpl_applied185/1 -> MinMax/186
  DFC_BattUNpl_applied186/1 -> MinMax/187
  DFC_BattUNpl_applied187/1 -> MinMax/188
  DFC_BattUNpl_applied188/1 -> MinMax/189
  DFC_BattUNpl_applied189/1 -> MinMax/190
  GaCFM_AFEComLost_flg/1 -> Data Type Conversion/1
  Data Type Conversion/1 -> Sum of Elements/1
  Data Type Conversion1/1 -> Sum of Elements1/1
  Data Type Conversion2/1 -> Sum of Elements2/1
  Data Type Conversion3/1 -> Sum of Elements3/1
  Data Type Conversion4/1 -> Sum of Elements4/1
  Data Type Conversion5/1 -> Sum of Elements5/1
  Data Type Conversion6/1 -> Sum of Elements6/1
  Data Type Conversion7/1 -> Sum of Elements7/1
  Data Type Conversion8/1 -> Sum of Elements8/1
  GaCFM_AFECellVoltUpdErr_flg/1 -> Data Type Conversion1/1
  GaCFM_AFECellTempUpdErr_flg/1 -> Data Type Conversion2/1
  GaCFM_AFESampleErr_flg/1 -> Data Type Conversion3/1
  GaCFM_AFECellVoltLineOpen_flg/1 -> Data Type Conversion4/1
  GaCFM_AFEGpioLineOpen_flg/1 -> Data Type Conversion5/1
  GaCFM_AFEAdcRelatedErr_flg/1 -> Data Type Conversion6/1
  GaCFM_AFEDiagModeExitErr_flg/1 -> Data Type Conversion7/1
  GaCFM_AFEOtherErr_flg/1 -> Data Type Conversion8/1
  Sum of Elements/1 -> Relational Operator1/1
  DFES_Cls_DFC_BattUNpl_C_zero190/1 -> Relational Operator1/2
  DFES_Cls_DFC_BattUNpl_C_zero191/1 -> Relational Operator2/2
  Relational Operator2/1 -> DFC_BattUNpl_applied182/2
  Sum of Elements1/1 -> Relational Operator2/1
  DFES_Cls_DFC_BattUNpl_C_zero192/1 -> Relational Operator3/2
  DFES_Cls_DFC_BattUNpl_C_zero193/1 -> Relational Operator4/2
  DFES_Cls_DFC_BattUNpl_C_zero194/1 -> Relational Operator5/2
  DFES_Cls_DFC_BattUNpl_C_zero195/1 -> Relational Operator6/2
  DFES_Cls_DFC_BattUNpl_C_zero196/1 -> Relational Operator7/2
  Sum of Elements2/1 -> Relational Operator3/1
  Sum of Elements3/1 -> Relational Operator4/1
  Sum of Elements4/1 -> Relational Operator5/1
  Sum of Elements5/1 -> Relational Operator6/1
  Sum of Elements6/1 -> Relational Operator7/1
  DFES_Cls_DFC_BattUNpl_C_zero197/1 -> Relational Operator8/2
  Sum of Elements7/1 -> Relational Operator8/1
  DFES_Cls_DFC_BattUNpl_C_zero198/1 -> Relational Operator9/2
  Sum of Elements8/1 -> Relational Operator9/1
  DFC_BattUNpl_182/1 -> DFC_BattUNpl_1_compare181/1
  DFC_BattUNpl_1_compare181/1 -> DFC_BattUNpl_applied190/2
  DFES_Cls_DFC_BattUNpl_C_zero199/1 -> DFC_BattUNpl_applied190/3
  DFC_BattUNpl_applied190/1 -> MinMax/191
  DFES_Cls_DFC_BattUNpl_C190/1 -> DFC_BattUNpl_applied190/1
  DFC_AcDischgFobd/1 -> DFC_BattUNpl_182/1
  DFC_BattUNpl_183/1 -> DFC_BattUNpl_1_compare182/1
  DFC_BattUNpl_1_compare182/1 -> DFC_BattUNpl_applied191/2
  DFES_Cls_DFC_BattUNpl_C_zero200/1 -> DFC_BattUNpl_applied191/3
  DFC_BattUNpl_184/1 -> DFC_BattUNpl_1_compare183/1
  DFC_BattUNpl_1_compare183/1 -> DFC_BattUNpl_applied192/2
  DFES_Cls_DFC_BattUNpl_C_zero201/1 -> DFC_BattUNpl_applied192/3
  DFC_BattUNpl_185/1 -> DFC_BattUNpl_1_compare184/1
  DFC_BattUNpl_1_compare184/1 -> DFC_BattUNpl_applied193/2
  DFES_Cls_DFC_BattUNpl_C_zero202/1 -> DFC_BattUNpl_applied193/3
  DFC_BattUNpl_186/1 -> DFC_BattUNpl_1_compare185/1
  DFC_BattUNpl_1_compare185/1 -> DFC_BattUNpl_applied194/2
  DFES_Cls_DFC_BattUNpl_C_zero203/1 -> DFC_BattUNpl_applied194/3
  DFC_BattUNpl_applied191/1 -> MinMax/192
  DFC_BattUNpl_applied192/1 -> MinMax/193
  DFC_BattUNpl_applied193/1 -> MinMax/194
  DFC_BattUNpl_applied194/1 -> MinMax/195
  DFES_Cls_DFC_BattUNpl_C191/1 -> DFC_BattUNpl_applied191/1
  DFES_Cls_DFC_BattUNpl_C192/1 -> DFC_BattUNpl_applied192/1
  DFES_Cls_DFC_BattUNpl_C193/1 -> DFC_BattUNpl_applied193/1
  DFES_Cls_DFC_BattUNpl_C194/1 -> DFC_BattUNpl_applied194/1
  DFC_BalCirOpenFlt/1 -> DFC_BattUNpl_183/1
  DFC_BalCirShortFlt/1 -> DFC_BattUNpl_184/1
  DFC_BalTempHighFlt/1 -> DFC_BattUNpl_185/1
  DFC_HVSmplComFlt/1 -> DFC_BattUNpl_186/1
  DFC_BattUNpl_187/1 -> DFC_BattUNpl_1_compare186/1
  DFC_BattUNpl_1_compare186/1 -> DFC_BattUNpl_applied195/2
  DFES_Cls_DFC_BattUNpl_C_zero204/1 -> DFC_BattUNpl_applied195/3
  DFES_Cls_DFC_BattUNpl_C195/1 -> DFC_BattUNpl_applied195/1
  DFC_BattUNpl_188/1 -> DFC_BattUNpl_1_compare187/1
  DFC_BattUNpl_1_compare187/1 -> DFC_BattUNpl_applied196/2
  DFES_Cls_DFC_BattUNpl_C_zero205/1 -> DFC_BattUNpl_applied196/3
  DFES_Cls_DFC_BattUNpl_C196/1 -> DFC_BattUNpl_applied196/1
  DFC_BattUNpl_189/1 -> DFC_BattUNpl_1_compare188/1
  DFC_BattUNpl_1_compare188/1 -> DFC_BattUNpl_applied197/2
  DFES_Cls_DFC_BattUNpl_C_zero206/1 -> DFC_BattUNpl_applied197/3
  DFES_Cls_DFC_BattUNpl_C197/1 -> DFC_BattUNpl_applied197/1
  DFC_BattUNpl_190/1 -> DFC_BattUNpl_1_compare189/1
  DFC_BattUNpl_1_compare189/1 -> DFC_BattUNpl_applied198/2
  DFES_Cls_DFC_BattUNpl_C_zero207/1 -> DFC_BattUNpl_applied198/3
  DFES_Cls_DFC_BattUNpl_C198/1 -> DFC_BattUNpl_applied198/1
  DFC_BattUNpl_191/1 -> DFC_BattUNpl_1_compare190/1
  DFC_BattUNpl_1_compare190/1 -> DFC_BattUNpl_applied199/2
  DFES_Cls_DFC_BattUNpl_C_zero208/1 -> DFC_BattUNpl_applied199/3
  DFES_Cls_DFC_BattUNpl_C199/1 -> DFC_BattUNpl_applied199/1
  DFC_BattUNpl_applied195/1 -> MinMax/196
  DFC_BattUNpl_applied196/1 -> MinMax/197
  DFC_BattUNpl_applied197/1 -> MinMax/198
  DFC_BattUNpl_applied198/1 -> MinMax/199
  DFC_BattUNpl_applied199/1 -> MinMax/200
  DFC_HVSmplSigErr/1 -> DFC_BattUNpl_187/1
  DFC_HVSmplSplyFlt/1 -> DFC_BattUNpl_188/1
  DFC_CABVoltOutOfRng/1 -> DFC_BattUNpl_189/1
  DFC_CABDevFlt/1 -> DFC_BattUNpl_190/1
  DFC_BMSSplyPwrAbnToLem/1 -> DFC_BattUNpl_191/1
  DFC_BattUNpl_192/1 -> DFC_BattUNpl_1_compare191/1
  DFC_BattUNpl_1_compare191/1 -> DFC_BattUNpl_applied200/2
  DFES_Cls_DFC_BattUNpl_C_zero209/1 -> DFC_BattUNpl_applied200/3
  DFES_Cls_DFC_BattUNpl_C200/1 -> DFC_BattUNpl_applied200/1
  DFC_BattUNpl_applied200/1 -> MinMax/201
  DFC_BattUNpl_193/1 -> DFC_BattUNpl_1_compare192/1
  DFC_BattUNpl_1_compare192/1 -> DFC_BattUNpl_applied201/2
  DFES_Cls_DFC_BattUNpl_C_zero210/1 -> DFC_BattUNpl_applied201/3
  DFC_BattUNpl_applied201/1 -> MinMax/202
  DFES_Cls_DFC_BattUNpl_C201/1 -> DFC_BattUNpl_applied201/1
  DFC_BattUNpl_194/1 -> DFC_BattUNpl_1_compare193/1
  DFC_BattUNpl_1_compare193/1 -> DFC_BattUNpl_applied202/2
  DFES_Cls_DFC_BattUNpl_C_zero211/1 -> DFC_BattUNpl_applied202/3
  DFES_Cls_DFC_BattUNpl_C202/1 -> DFC_BattUNpl_applied202/1
  DFC_BattUNpl_195/1 -> DFC_BattUNpl_1_compare194/1
  DFC_BattUNpl_1_compare194/1 -> DFC_BattUNpl_applied203/2
  DFES_Cls_DFC_BattUNpl_C_zero212/1 -> DFC_BattUNpl_applied203/3
  DFES_Cls_DFC_BattUNpl_C203/1 -> DFC_BattUNpl_applied203/1
  DFC_BattUNpl_applied202/1 -> MinMax/203
  DFC_BattUNpl_applied203/1 -> MinMax/204
  DFC_BattUNpl_196/1 -> DFC_BattUNpl_1_compare195/1
  DFC_BattUNpl_1_compare195/1 -> DFC_BattUNpl_applied204/2
  DFES_Cls_DFC_BattUNpl_C_zero213/1 -> DFC_BattUNpl_applied204/3
  DFC_BattUNpl_197/1 -> DFC_BattUNpl_1_compare196/1
  DFC_BattUNpl_1_compare196/1 -> DFC_BattUNpl_applied205/2
  DFES_Cls_DFC_BattUNpl_C_zero214/1 -> DFC_BattUNpl_applied205/3
  DFES_Cls_DFC_BattUNpl_C205/1 -> DFC_BattUNpl_applied205/1
  DFC_BattUNpl_198/1 -> DFC_BattUNpl_1_compare197/1
  DFC_BattUNpl_1_compare197/1 -> DFC_BattUNpl_applied206/2
  DFES_Cls_DFC_BattUNpl_C_zero215/1 -> DFC_BattUNpl_applied206/3
  DFC_BattUNpl_199/1 -> DFC_BattUNpl_1_compare198/1
  DFC_BattUNpl_1_compare198/1 -> DFC_BattUNpl_applied207/2
  DFES_Cls_DFC_BattUNpl_C_zero216/1 -> DFC_BattUNpl_applied207/3
  DFES_Cls_DFC_BattUNpl_C207/1 -> DFC_BattUNpl_applied207/1
  DFC_BattUNpl_200/1 -> DFC_BattUNpl_1_compare199/1
  DFC_BattUNpl_1_compare199/1 -> DFC_BattUNpl_applied208/2
  DFES_Cls_DFC_BattUNpl_C_zero217/1 -> DFC_BattUNpl_applied208/3
  DFC_BattUNpl_201/1 -> DFC_BattUNpl_1_compare200/1
  DFC_BattUNpl_1_compare200/1 -> DFC_BattUNpl_applied209/2
  DFES_Cls_DFC_BattUNpl_C_zero218/1 -> DFC_BattUNpl_applied209/3
  DFES_Cls_DFC_BattUNpl_C209/1 -> DFC_BattUNpl_applied209/1
  DFC_BattUNpl_202/1 -> DFC_BattUNpl_1_compare201/1
  DFC_BattUNpl_1_compare201/1 -> DFC_BattUNpl_applied210/2
  DFES_Cls_DFC_BattUNpl_C_zero219/1 -> DFC_BattUNpl_applied210/3
  DFC_BattUNpl_203/1 -> DFC_BattUNpl_1_compare202/1
  DFC_BattUNpl_1_compare202/1 -> DFC_BattUNpl_applied211/2
  DFES_Cls_DFC_BattUNpl_C_zero220/1 -> DFC_BattUNpl_applied211/3
  DFES_Cls_DFC_BattUNpl_C211/1 -> DFC_BattUNpl_applied211/1
  DFC_BattUNpl_applied204/1 -> MinMax/205
  DFC_BattUNpl_applied205/1 -> MinMax/206
  DFC_BattUNpl_applied208/1 -> MinMax/209
  DFC_BattUNpl_applied209/1 -> MinMax/210
  DFC_BattUNpl_applied206/1 -> MinMax/207
  DFC_BattUNpl_applied207/1 -> MinMax/208
  DFC_BattUNpl_applied211/1 -> MinMax/212
  DFC_BattUNpl_applied210/1 -> MinMax/211
  DFES_Cls_DFC_BattUNpl_C206/1 -> DFC_BattUNpl_applied206/1
  DFES_Cls_DFC_BattUNpl_C208/1 -> DFC_BattUNpl_applied208/1
  DFES_Cls_DFC_BattUNpl_C210/1 -> DFC_BattUNpl_applied210/1
  DFES_Cls_DFC_BattUNpl_C204/1 -> DFC_BattUNpl_applied204/1
  DFC_BattUNpl_204/1 -> DFC_BattUNpl_1_compare203/1
  DFC_BattUNpl_1_compare203/1 -> DFC_BattUNpl_applied212/2
  DFES_Cls_DFC_BattUNpl_C_zero221/1 -> DFC_BattUNpl_applied212/3
  DFC_BattUNpl_205/1 -> DFC_BattUNpl_1_compare204/1
  DFC_BattUNpl_1_compare204/1 -> DFC_BattUNpl_applied213/2
  DFES_Cls_DFC_BattUNpl_C_zero222/1 -> DFC_BattUNpl_applied213/3
  DFES_Cls_DFC_BattUNpl_C212/1 -> DFC_BattUNpl_applied213/1
  DFC_BattUNpl_applied212/1 -> MinMax/213
  DFC_BattUNpl_applied213/1 -> MinMax/214
  DFES_Cls_DFC_BattUNpl_C213/1 -> DFC_BattUNpl_applied212/1
  DFC_BMSSplyPwrAbnToCAB/1 -> DFC_BattUNpl_192/1
  DFC_NVMReadError/1 -> DFC_BattUNpl_193/1
  DFC_KL30Shutdown/1 -> DFC_BattUNpl_194/1
  DFC_MCUResetFlt/1 -> DFC_BattUNpl_195/1
  DFC_BattSohChk/1 -> DFC_BattUNpl_196/1
  DFC_CalCANBusOff/1 -> DFC_BattUNpl_197/1
  DFC_ThmRnwyWarn/1 -> DFC_BattUNpl_198/1
  DFC_PchgOvrCurrFlt/1 -> DFC_BattUNpl_199/1
  DFC_SBCSplyPwrOvrVolt/1 -> DFC_BattUNpl_200/1
  DFC_SBCSplyPwrUnderVolt/1 -> DFC_BattUNpl_201/1
  DFC_SBCSplyPwrOvrCurr/1 -> DFC_BattUNpl_202/1
  DFC_CrashChkHwFrqAbnorm/1 -> DFC_BattUNpl_203/1
  DFC_CrashChkHwDutyAbnorm/1 -> DFC_BattUNpl_204/1
  DFC_AFETempHighFlt/1 -> DFC_BattUNpl_205/1
  DFC_BattUNpl_206/1 -> DFC_BattUNpl_1_compare205/1
  DFC_EVCCDevFlt/1 -> DFC_BattUNpl_206/1
  DFC_BattUNpl_207/1 -> DFC_BattUNpl_1_compare206/1
  DFC_BattUNpl_208/1 -> DFC_BattUNpl_1_compare207/1
  DFC_BattUNpl_209/1 -> DFC_BattUNpl_1_compare208/1
  DFC_BattUNpl_210/1 -> DFC_BattUNpl_1_compare209/1
  DFC_BattUNpl_211/1 -> DFC_BattUNpl_1_compare210/1
  DFC_EVCCSplyPwrFlt/1 -> DFC_BattUNpl_207/1
  DFC_EVCCVehComFlt/1 -> DFC_BattUNpl_208/1
  DFC_EVCCPileComFlt/1 -> DFC_BattUNpl_209/1
  DFC_EVCCVehHwFlt/1 -> DFC_BattUNpl_210/1
  DFC_EVCCPileHwFlt/1 -> DFC_BattUNpl_211/1
  DFC_BattUNpl_1_compare205/1 -> Logical Operator/1
  DFC_BattUNpl_1_compare208/1 -> Logical Operator/4
  DFC_BattUNpl_1_compare206/1 -> Logical Operator/2
  DFC_BattUNpl_1_compare209/1 -> Logical Operator/5
  DFC_BattUNpl_1_compare207/1 -> Logical Operator/3
  DFC_BattUNpl_1_compare210/1 -> Logical Operator/6
  Logical Operator/1 -> DFC_BattUNpl_applied214/2
  DFES_Cls_DFC_BattUNpl_C_zero223/1 -> DFC_BattUNpl_applied214/3
  DFES_Cls_DFC_BattUNpl_C214/1 -> DFC_BattUNpl_applied214/1
  DFC_BattUNpl_213/1 -> DFC_BattUNpl_1_compare212/1
  DFC_IsoS1SwStuckOpen/1 -> DFC_BattUNpl_213/1
  DFC_BattUNpl_214/1 -> DFC_BattUNpl_1_compare213/1
  DFC_BattUNpl_215/1 -> DFC_BattUNpl_1_compare214/1
  DFC_BattUNpl_216/1 -> DFC_BattUNpl_1_compare215/1
  DFC_BattUNpl_217/1 -> DFC_BattUNpl_1_compare216/1
  DFC_BattUNpl_218/1 -> DFC_BattUNpl_1_compare217/1
  DFC_IsoS1SwStuckClsd/1 -> DFC_BattUNpl_214/1
  DFC_IsoS2SwStuckOpen/1 -> DFC_BattUNpl_215/1
  DFC_IsoS2SwStuckClsd/1 -> DFC_BattUNpl_216/1
  DFC_IsoS3SwStuckOpen/1 -> DFC_BattUNpl_217/1
  DFC_IsoS3SwStuckClsd/1 -> DFC_BattUNpl_218/1
  DFC_BattUNpl_1_compare212/1 -> Logical Operator1/1
  DFC_BattUNpl_1_compare213/1 -> Logical Operator1/2
  DFC_BattUNpl_1_compare214/1 -> Logical Operator1/3
  DFC_BattUNpl_1_compare215/1 -> Logical Operator1/4
  DFC_BattUNpl_1_compare216/1 -> Logical Operator1/5
  DFC_BattUNpl_1_compare217/1 -> Logical Operator1/6
  Logical Operator1/1 -> DFC_BattUNpl_applied215/2
  DFES_Cls_DFC_BattUNpl_C_zero224/1 -> DFC_BattUNpl_applied215/3
  DFES_Cls_DFC_BattUNpl_C215/1 -> DFC_BattUNpl_applied215/1
  DFC_BattUNpl_212/1 -> DFC_BattUNpl_1_compare211/1
  DFC_BattUNpl_1_compare211/1 -> DFC_BattUNpl_applied216/2
  DFES_Cls_DFC_BattUNpl_C_zero225/1 -> DFC_BattUNpl_applied216/3
  DFC_BattUNpl_219/1 -> DFC_BattUNpl_1_compare218/1
  DFC_BattUNpl_1_compare218/1 -> DFC_BattUNpl_applied217/2
  DFES_Cls_DFC_BattUNpl_C_zero226/1 -> DFC_BattUNpl_applied217/3
  DFC_AFEResetFlt/1 -> DFC_BattUNpl_212/1
  DFC_AFESplyFlt/1 -> DFC_BattUNpl_219/1
  DFC_BattUNpl_220/1 -> DFC_BattUNpl_1_compare219/1
  DFC_BattUNpl_221/1 -> DFC_BattUNpl_1_compare220/1
  DFC_BattUNpl_222/1 -> DFC_BattUNpl_1_compare221/1
  DFC_BattUNpl_223/1 -> DFC_BattUNpl_1_compare222/1
  DFC_PreHeatPtcErr/1 -> DFC_BattUNpl_223/1
  DFC_PreHeatObcStatusErr/1 -> DFC_BattUNpl_222/1
  DFC_PreHeatVcuReqTmt/1 -> DFC_BattUNpl_221/1
  DFC_PreHeatErr/1 -> DFC_BattUNpl_220/1
  DFC_BattUNpl_1_compare219/1 -> Logical Operator2/1
  DFC_BattUNpl_1_compare220/1 -> Logical Operator2/2
  DFC_BattUNpl_1_compare221/1 -> Logical Operator2/3
  DFC_BattUNpl_1_compare222/1 -> Logical Operator2/4
  Logical Operator2/1 -> DFC_BattUNpl_applied218/2
  DFES_Cls_DFC_BattUNpl_C_zero227/1 -> DFC_BattUNpl_applied218/3
  DFES_Cls_DFC_BattUNpl_C218/1 -> DFC_BattUNpl_applied218/1
  DFC_BattUNpl_224/1 -> DFC_BattUNpl_1_compare223/1
  DFC_BattUNpl_225/1 -> DFC_BattUNpl_1_compare224/1
  DFC_BattUNpl_226/1 -> DFC_BattUNpl_1_compare225/1
  DFC_BattUNpl_227/1 -> DFC_BattUNpl_1_compare226/1
  DFC_BattUNpl_1_compare223/1 -> Logical Operator3/1
  DFC_BattUNpl_1_compare224/1 -> Logical Operator3/2
  DFC_BattUNpl_1_compare225/1 -> Logical Operator3/3
  DFC_BattUNpl_1_compare226/1 -> Logical Operator3/4
  DFC_MPosRlyDrvScb/1 -> DFC_BattUNpl_224/1
  DFC_MPosRlyDrvScg/1 -> DFC_BattUNpl_225/1
  DFC_MPosRlyDrvOL/1 -> DFC_BattUNpl_226/1
  DFC_MposRlyDrvOvrCurr/1 -> DFC_BattUNpl_227/1
  DFC_BattUNpl_228/1 -> DFC_BattUNpl_1_compare227/1
  DFC_BattUNpl_1_compare227/1 -> Logical Operator3/5
  DFC_MPosRlyDrvFault/1 -> DFC_BattUNpl_228/1
  Logical Operator3/1 -> DFC_BattUNpl_applied219/2
  DFES_Cls_DFC_BattUNpl_C_zero228/1 -> DFC_BattUNpl_applied219/3
  DFES_Cls_DFC_BattUNpl_C219/1 -> DFC_BattUNpl_applied219/1
  DFC_BattUNpl_229/1 -> DFC_BattUNpl_1_compare228/1
  DFC_BattUNpl_230/1 -> DFC_BattUNpl_1_compare229/1
  DFC_BattUNpl_231/1 -> DFC_BattUNpl_1_compare230/1
  DFC_BattUNpl_232/1 -> DFC_BattUNpl_1_compare231/1
  DFC_BattUNpl_1_compare228/1 -> Logical Operator4/1
  DFC_BattUNpl_1_compare229/1 -> Logical Operator4/2
  DFC_BattUNpl_1_compare230/1 -> Logical Operator4/3
  DFC_BattUNpl_1_compare231/1 -> Logical Operator4/4
  DFC_BattUNpl_233/1 -> DFC_BattUNpl_1_compare232/1
  DFC_BattUNpl_1_compare232/1 -> Logical Operator4/5
  DFC_MNegRlyDrvScb/1 -> DFC_BattUNpl_229/1
  DFC_MNegRlyDrvScg/1 -> DFC_BattUNpl_230/1
  DFC_MNegRlyDrvOL/1 -> DFC_BattUNpl_231/1
  DFC_MNegRlyDrvOvrCurr/1 -> DFC_BattUNpl_232/1
  DFC_MNegRlyDrvFault/1 -> DFC_BattUNpl_233/1
  Logical Operator4/1 -> DFC_BattUNpl_applied220/2
  DFES_Cls_DFC_BattUNpl_C_zero229/1 -> DFC_BattUNpl_applied220/3
  DFES_Cls_DFC_BattUNpl_C220/1 -> DFC_BattUNpl_applied220/1
  DFC_BattUNpl_234/1 -> DFC_BattUNpl_1_compare233/1
  DFC_BattUNpl_235/1 -> DFC_BattUNpl_1_compare234/1
  DFC_BattUNpl_236/1 -> DFC_BattUNpl_1_compare235/1
  DFC_BattUNpl_237/1 -> DFC_BattUNpl_1_compare236/1
  DFC_BattUNpl_1_compare233/1 -> Logical Operator5/1
  DFC_BattUNpl_1_compare234/1 -> Logical Operator5/2
  DFC_BattUNpl_1_compare235/1 -> Logical Operator5/3
  DFC_BattUNpl_1_compare236/1 -> Logical Operator5/4
  DFC_BattUNpl_238/1 -> DFC_BattUNpl_1_compare237/1
  DFC_BattUNpl_1_compare237/1 -> Logical Operator5/5
  Logical Operator5/1 -> DFC_BattUNpl_applied221/2
  DFES_Cls_DFC_BattUNpl_C_zero230/1 -> DFC_BattUNpl_applied221/3
  DFES_Cls_DFC_BattUNpl_C221/1 -> DFC_BattUNpl_applied221/1
  DFC_DcPosRlyDrvScb/1 -> DFC_BattUNpl_234/1
  DFC_DcPosRlyDrvScg/1 -> DFC_BattUNpl_235/1
  DFC_DcPosRlyDrvOL/1 -> DFC_BattUNpl_236/1
  DFC_DChrgPosRlyDrvOvrCurr/1 -> DFC_BattUNpl_237/1
  DFC_DcPosRlyDrvFault/1 -> DFC_BattUNpl_238/1
  DFC_BattUNpl_239/1 -> DFC_BattUNpl_1_compare238/1
  DFC_BattUNpl_240/1 -> DFC_BattUNpl_1_compare239/1
  DFC_BattUNpl_241/1 -> DFC_BattUNpl_1_compare240/1
  DFC_BattUNpl_242/1 -> DFC_BattUNpl_1_compare241/1
  DFC_BattUNpl_1_compare238/1 -> Logical Operator6/1
  DFC_BattUNpl_1_compare239/1 -> Logical Operator6/2
  DFC_BattUNpl_1_compare240/1 -> Logical Operator6/3
  DFC_BattUNpl_1_compare241/1 -> Logical Operator6/4
  DFC_BattUNpl_243/1 -> DFC_BattUNpl_1_compare242/1
  DFC_BattUNpl_1_compare242/1 -> Logical Operator6/5
  Logical Operator6/1 -> DFC_BattUNpl_applied222/2
  DFES_Cls_DFC_BattUNpl_C_zero231/1 -> DFC_BattUNpl_applied222/3
  DFES_Cls_DFC_BattUNpl_C222/1 -> DFC_BattUNpl_applied222/1
  DFC_DcNegRlyDrvScb/1 -> DFC_BattUNpl_239/1
  DFC_DcNegRlyDrvScg/1 -> DFC_BattUNpl_240/1
  DFC_DcNegRlyDrvOL/1 -> DFC_BattUNpl_241/1
  DFC_DChrgNegRlyDrvOvrCurr/1 -> DFC_BattUNpl_242/1
  DFC_DcNegRlyDrvFault/1 -> DFC_BattUNpl_243/1
  DFC_BattUNpl_244/1 -> DFC_BattUNpl_1_compare243/1
  DFC_BattUNpl_245/1 -> DFC_BattUNpl_1_compare244/1
  DFC_BattUNpl_246/1 -> DFC_BattUNpl_1_compare245/1
  DFC_BattUNpl_247/1 -> DFC_BattUNpl_1_compare246/1
  DFC_BattUNpl_1_compare243/1 -> Logical Operator7/1
  DFC_BattUNpl_1_compare244/1 -> Logical Operator7/2
  DFC_BattUNpl_1_compare245/1 -> Logical Operator7/3
  DFC_BattUNpl_1_compare246/1 -> Logical Operator7/4
  Logical Operator7/1 -> DFC_BattUNpl_applied223/2
  DFES_Cls_DFC_BattUNpl_C_zero232/1 -> DFC_BattUNpl_applied223/3
  DFES_Cls_DFC_BattUNpl_C223/1 -> DFC_BattUNpl_applied223/1
  DFC_PreRlyDrvScb/1 -> DFC_BattUNpl_244/1
  DFC_PreRlyDrvOL/1 -> DFC_BattUNpl_246/1
  DFC_PreRlyDrvScg/1 -> DFC_BattUNpl_245/1
  DFC_PrRlyDrvOvrCurr/1 -> DFC_BattUNpl_247/1
  DFES_Cls_DFC_BattUNpl_C216/1 -> DFC_BattUNpl_applied216/1
  DFES_Cls_DFC_BattUNpl_C217/1 -> DFC_BattUNpl_applied217/1
  DFC_BattUNpl_applied216/1 -> MinMax/215
  DFC_BattUNpl_applied217/1 -> MinMax/216
  DFC_BattUNpl_248/1 -> DFC_BattUNpl_1_compare247/1
  DFC_BattUNpl_1_compare247/1 -> DFC_BattUNpl_applied224/2
  DFES_Cls_DFC_BattUNpl_C224/1 -> DFC_BattUNpl_applied224/1
  DFES_Cls_DFC_BattUNpl_C_zero233/1 -> DFC_BattUNpl_applied224/3
  DFC_CellTAlrmMax/1 -> DFC_BattUNpl_248/1
  DFC_BattUNpl_249/1 -> DFC_BattUNpl_1_compare248/1
  DFC_BattUNpl_1_compare248/1 -> DFC_BattUNpl_applied225/2
  DFES_Cls_DFC_BattUNpl_C225/1 -> DFC_BattUNpl_applied225/1
  DFES_Cls_DFC_BattUNpl_C_zero234/1 -> DFC_BattUNpl_applied225/3
  DFC_CellTFaultMax/1 -> DFC_BattUNpl_249/1
  DFC_BattUNpl_250/1 -> DFC_BattUNpl_1_compare249/1
  DFC_BattUNpl_1_compare249/1 -> DFC_BattUNpl_applied226/2
  DFES_Cls_DFC_BattUNpl_C226/1 -> DFC_BattUNpl_applied226/1
  DFES_Cls_DFC_BattUNpl_C_zero235/1 -> DFC_BattUNpl_applied226/3
  DFC_CellTAlrmMin/1 -> DFC_BattUNpl_250/1
  DFC_BattUNpl_251/1 -> DFC_BattUNpl_1_compare250/1
  DFC_BattUNpl_1_compare250/1 -> DFC_BattUNpl_applied227/2
  DFES_Cls_DFC_BattUNpl_C227/1 -> DFC_BattUNpl_applied227/1
  DFES_Cls_DFC_BattUNpl_C_zero236/1 -> DFC_BattUNpl_applied227/3
  DFC_CellTFaultMin/1 -> DFC_BattUNpl_251/1
  DFC_BattUNpl_252/1 -> DFC_BattUNpl_1_compare251/1
  DFC_BattUNpl_1_compare251/1 -> DFC_BattUNpl_applied228/2
  DFES_Cls_DFC_BattUNpl_C228/1 -> DFC_BattUNpl_applied228/1
  DFES_Cls_DFC_BattUNpl_C_zero237/1 -> DFC_BattUNpl_applied228/3
  DFC_CellTempVldMin/1 -> DFC_BattUNpl_252/1
  DFC_BattUNpl_253/1 -> DFC_BattUNpl_1_compare252/1
  DFC_BattUNpl_1_compare252/1 -> DFC_BattUNpl_applied229/2
  DFES_Cls_DFC_BattUNpl_C229/1 -> DFC_BattUNpl_applied229/1
  DFES_Cls_DFC_BattUNpl_C_zero238/1 -> DFC_BattUNpl_applied229/3
  DFC_CellTCnstMax/1 -> DFC_BattUNpl_253/1
  DFC_BattUNpl_254/1 -> DFC_BattUNpl_1_compare253/1
  DFC_BattUNpl_1_compare253/1 -> DFC_BattUNpl_applied230/2
  DFES_Cls_DFC_BattUNpl_C230/1 -> DFC_BattUNpl_applied230/1
  DFC_CellTGradtMax/1 -> DFC_BattUNpl_254/1
  DFC_BattUNpl_255/1 -> DFC_BattUNpl_1_compare254/1
  DFC_BattUNpl_1_compare254/1 -> DFC_BattUNpl_applied231/2
  DFES_Cls_DFC_BattUNpl_C231/1 -> DFC_BattUNpl_applied231/1
  DFES_Cls_DFC_BattUNpl_C_zero240/1 -> DFC_BattUNpl_applied231/3
  DFC_CellTWarnMax/1 -> DFC_BattUNpl_255/1
  DFC_BattUNpl_256/1 -> DFC_BattUNpl_1_compare255/1
  DFC_BattUNpl_1_compare255/1 -> DFC_BattUNpl_applied232/2
  DFES_Cls_DFC_BattUNpl_C232/1 -> DFC_BattUNpl_applied232/1
  DFES_Cls_DFC_BattUNpl_C_zero241/1 -> DFC_BattUNpl_applied232/3
  DFC_CellTWarnMin/1 -> DFC_BattUNpl_256/1
  DFC_BattUNpl_257/1 -> DFC_BattUNpl_1_compare256/1
  DFC_BattUNpl_1_compare256/1 -> DFC_BattUNpl_applied233/2
  DFES_Cls_DFC_BattUNpl_C233/1 -> DFC_BattUNpl_applied233/1
  DFES_Cls_DFC_BattUNpl_C_zero242/1 -> DFC_BattUNpl_applied233/3
  DFC_CellTempVldMax/1 -> DFC_BattUNpl_257/1
  DFC_BattUNpl_258/1 -> DFC_BattUNpl_1_compare257/1
  DFC_BattUNpl_1_compare257/1 -> DFC_BattUNpl_applied234/2
  DFES_Cls_DFC_BattUNpl_C234/1 -> DFC_BattUNpl_applied234/1
  DFES_Cls_DFC_BattUNpl_C_zero243/1 -> DFC_BattUNpl_applied234/3
  DFC_CellTHopMax/1 -> DFC_BattUNpl_258/1
  DFC_BattUNpl_applied224/1 -> MinMax/217
  DFC_BattUNpl_applied225/1 -> MinMax/218
  DFC_BattUNpl_applied226/1 -> MinMax/219
  DFC_BattUNpl_applied227/1 -> MinMax/220
  DFC_BattUNpl_applied228/1 -> MinMax/221
  DFC_BattUNpl_applied229/1 -> MinMax/222
  DFC_BattUNpl_applied230/1 -> MinMax/223
  DFC_BattUNpl_applied234/1 -> MinMax/227
  DFC_BattUNpl_applied233/1 -> MinMax/226
  DFC_BattUNpl_applied232/1 -> MinMax/225
  DFC_BattUNpl_applied231/1 -> MinMax/224
  DFES_Cls_DFC_BattUNpl_C_zero239/1 -> DFC_BattUNpl_applied230/3
  DFC_BattUNpl_applied214/1 -> MinMax/228
  DFC_BattUNpl_applied215/1 -> MinMax/229
  DFC_BattUNpl_applied218/1 -> MinMax/230
  DFC_BattUNpl_applied219/1 -> MinMax/231
  DFC_BattUNpl_applied220/1 -> MinMax/232
  DFC_BattUNpl_applied221/1 -> MinMax/233
  DFC_BattUNpl_applied222/1 -> MinMax/234
  DFC_BattUNpl_applied223/1 -> MinMax/235
  DFES_Cls_DFC_BattUNpl_C_zero244/1 -> DFC_BattUNpl_applied235/3
  DFC_BattUNpl_1_compare258/1 -> DFC_BattUNpl_applied235/2
  DFES_Cls_DFC_BattUNpl_C235/1 -> DFC_BattUNpl_applied235/1
  DFC_BattUNpl_259/1 -> DFC_BattUNpl_1_compare258/1
  DFC_TwoCurrSnsrFlt/1 -> DFC_BattUNpl_259/1
  DFES_Cls_DFC_BattUNpl_C_zero245/1 -> DFC_BattUNpl_applied236/3
  DFC_BattUNpl_260/1 -> DFC_BattUNpl_1_compare259/1
  DFES_Cls_DFC_BattUNpl_C236/1 -> DFC_BattUNpl_applied236/1
  DFC_BattUNpl_1_compare259/1 -> DFC_BattUNpl_applied236/2
  DFC_ThmRnwyAlarm/1 -> DFC_BattUNpl_260/1
  DFC_BattUNpl_applied235/1 -> MinMax/236
  DFC_BattUNpl_applied236/1 -> MinMax/237
  DFC_ChkSumMsg2A5Err/1 -> DFC_BattUNpl_261/1
  DFC_BattUNpl_1_compare260/1 -> DFC_BattUNpl_applied237/2
  DFES_Cls_DFC_BattUNpl_C237/1 -> DFC_BattUNpl_applied237/1
  DFC_BattUNpl_261/1 -> DFC_BattUNpl_1_compare260/1
  DFES_Cls_DFC_BattUNpl_C_zero246/1 -> DFC_BattUNpl_applied237/3
  DFES_Cls_DFC_BattUNpl_C_zero247/1 -> DFC_BattUNpl_applied238/3
  DFC_BattUNpl_262/1 -> DFC_BattUNpl_1_compare261/1
  DFES_Cls_DFC_BattUNpl_C238/1 -> DFC_BattUNpl_applied238/1
  DFC_BattUNpl_1_compare261/1 -> DFC_BattUNpl_applied238/2
  DFC_ChkSumMsg2A7Err/1 -> DFC_BattUNpl_262/1
  DFC_DchrgIsoChkLv1/1 -> DFC_BattUNpl_263/1
  DFC_BattUNpl_1_compare262/1 -> DFC_BattUNpl_applied239/2
  DFES_Cls_DFC_BattUNpl_C239/1 -> DFC_BattUNpl_applied239/1
  DFC_BattUNpl_263/1 -> DFC_BattUNpl_1_compare262/1
  DFES_Cls_DFC_BattUNpl_C_zero248/1 -> DFC_BattUNpl_applied239/3
  DFES_Cls_DFC_BattUNpl_C_zero249/1 -> DFC_BattUNpl_applied240/3
  DFC_BattUNpl_264/1 -> DFC_BattUNpl_1_compare263/1
  DFES_Cls_DFC_BattUNpl_C240/1 -> DFC_BattUNpl_applied240/1
  DFC_BattUNpl_1_compare263/1 -> DFC_BattUNpl_applied240/2
  DFC_DchrgIsoChkLv2/1 -> DFC_BattUNpl_264/1
  DFC_HVOffIsoChkLv1/1 -> DFC_BattUNpl_265/1
  DFC_BattUNpl_1_compare264/1 -> DFC_BattUNpl_applied241/2
  DFC_BattUNpl_265/1 -> DFC_BattUNpl_1_compare264/1
  DFES_Cls_DFC_BattUNpl_C_zero250/1 -> DFC_BattUNpl_applied241/3
  DFES_Cls_DFC_BattUNpl_C_zero251/1 -> DFC_BattUNpl_applied242/3
  DFC_BattUNpl_266/1 -> DFC_BattUNpl_1_compare265/1
  DFC_BattUNpl_1_compare265/1 -> DFC_BattUNpl_applied242/2
  DFC_HVOffIsoChkLv2/1 -> DFC_BattUNpl_266/1
  DFES_Cls_DFC_BattUNpl_C241/1 -> DFC_BattUNpl_applied241/1
  DFES_Cls_DFC_BattUNpl_C242/1 -> DFC_BattUNpl_applied242/1
  DFC_BattUNpl_applied237/1 -> MinMax/238
  DFC_BattUNpl_applied238/1 -> MinMax/239
  DFC_BattUNpl_applied239/1 -> MinMax/240
  DFC_BattUNpl_applied240/1 -> MinMax/241
  DFC_BattUNpl_applied241/1 -> MinMax/242
  DFC_BattUNpl_applied242/1 -> MinMax/243
  DFC_BattUNpl_applied243/1 -> MinMax/244
  DFES_Cls_DFC_BattUNpl_C243/1 -> DFC_BattUNpl_applied243/1
  DFC_BattUNpl_1_compare266/1 -> DFC_BattUNpl_applied243/2
  DFC_BattUNpl_267/1 -> DFC_BattUNpl_1_compare266/1
  DFES_Cls_DFC_BattUNpl_C_zero252/1 -> DFC_BattUNpl_applied243/3
  DFC_PackCrntSaf/1 -> DFC_BattUNpl_267/1
